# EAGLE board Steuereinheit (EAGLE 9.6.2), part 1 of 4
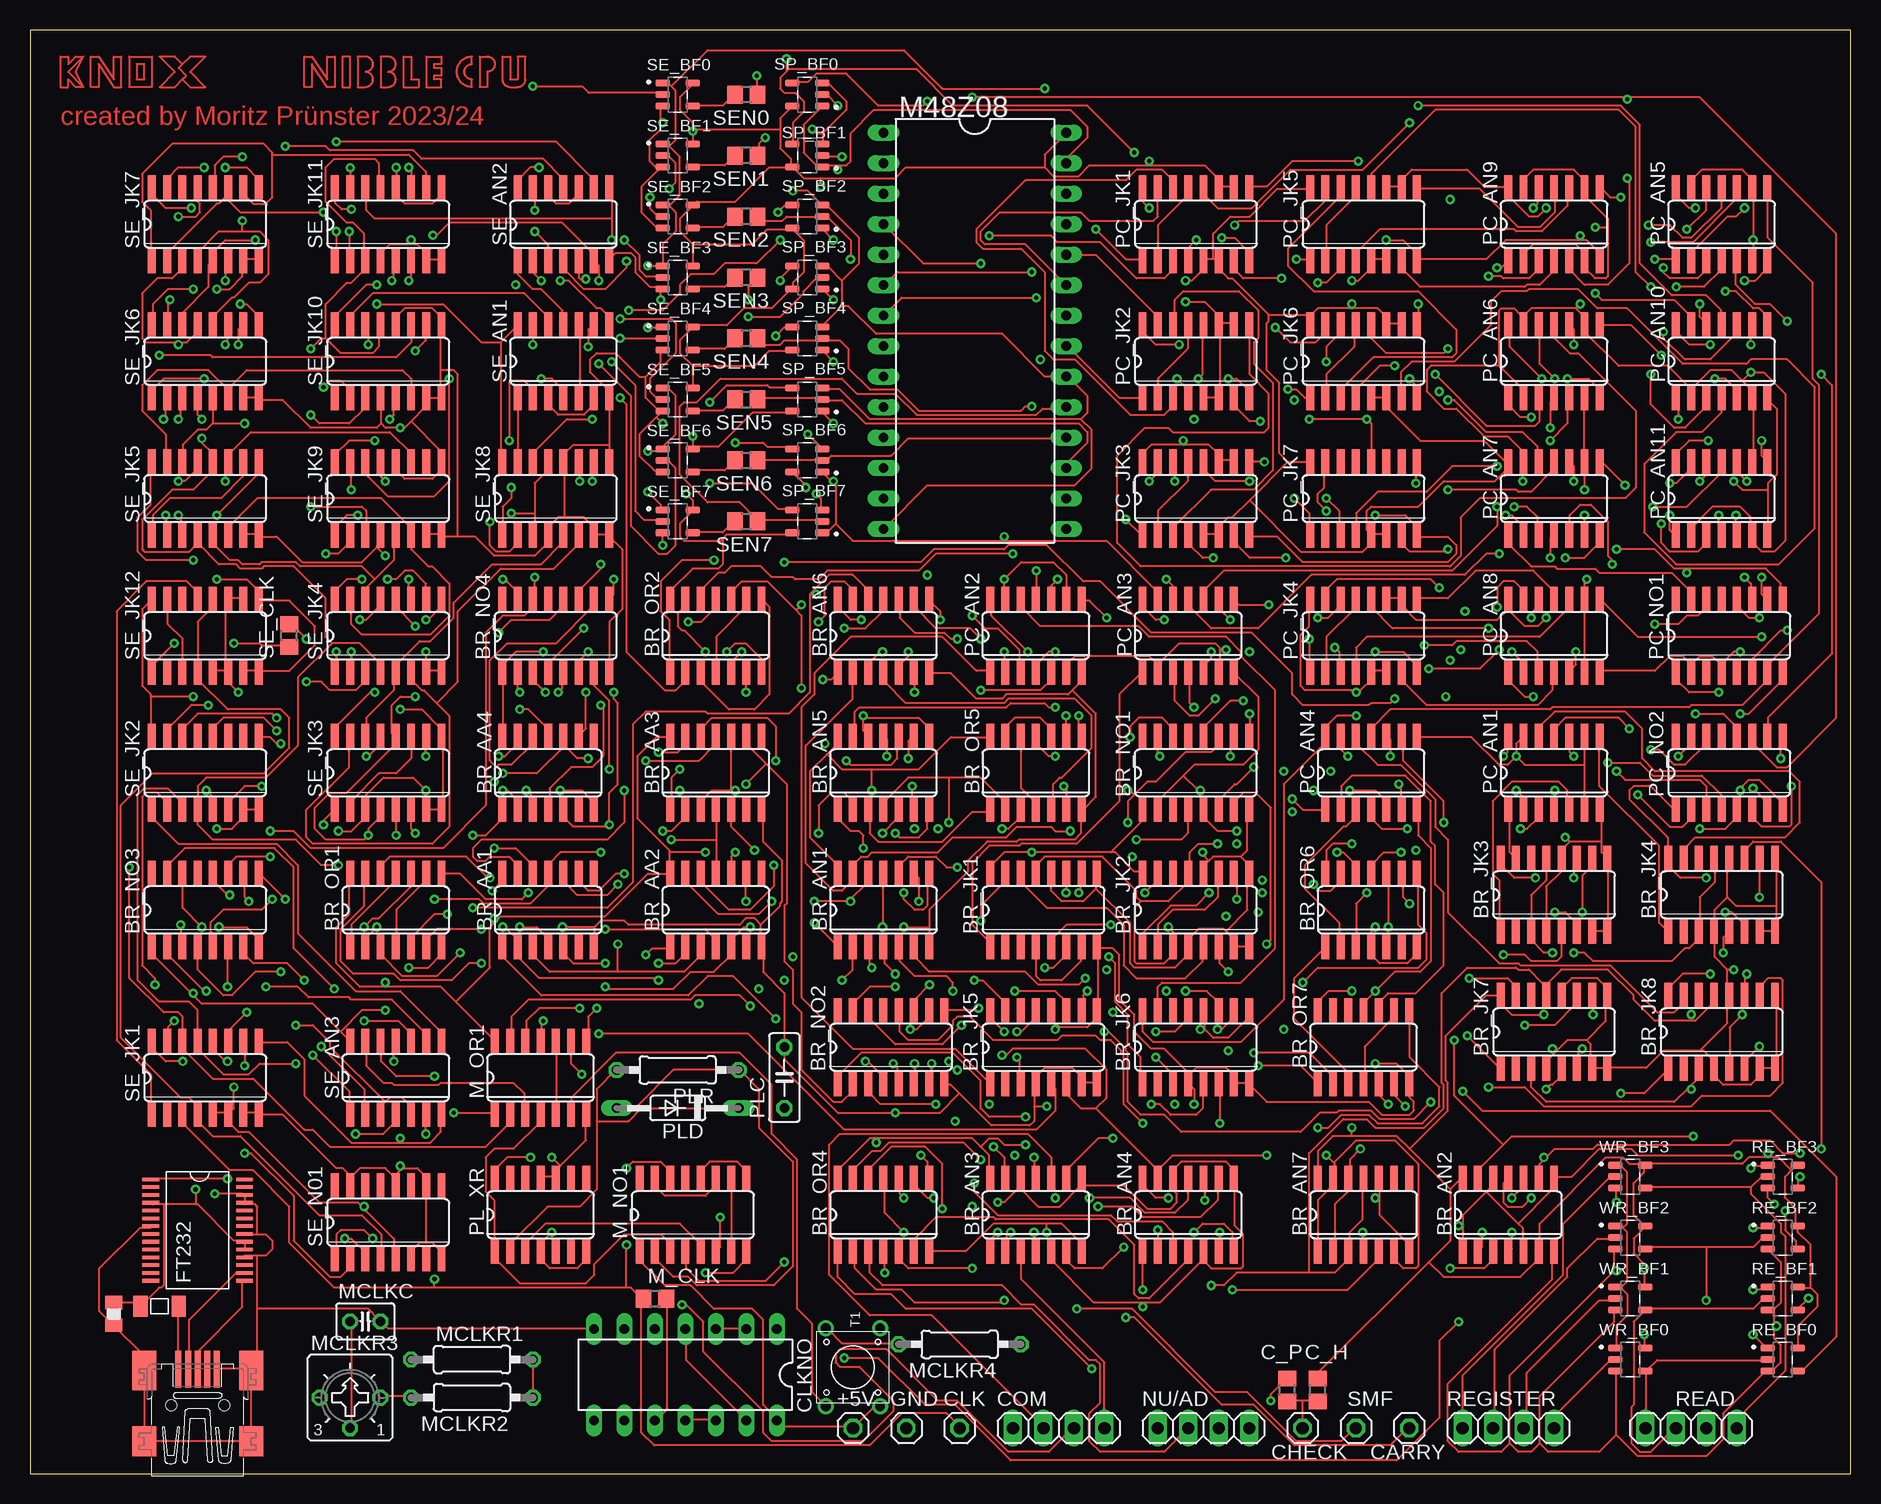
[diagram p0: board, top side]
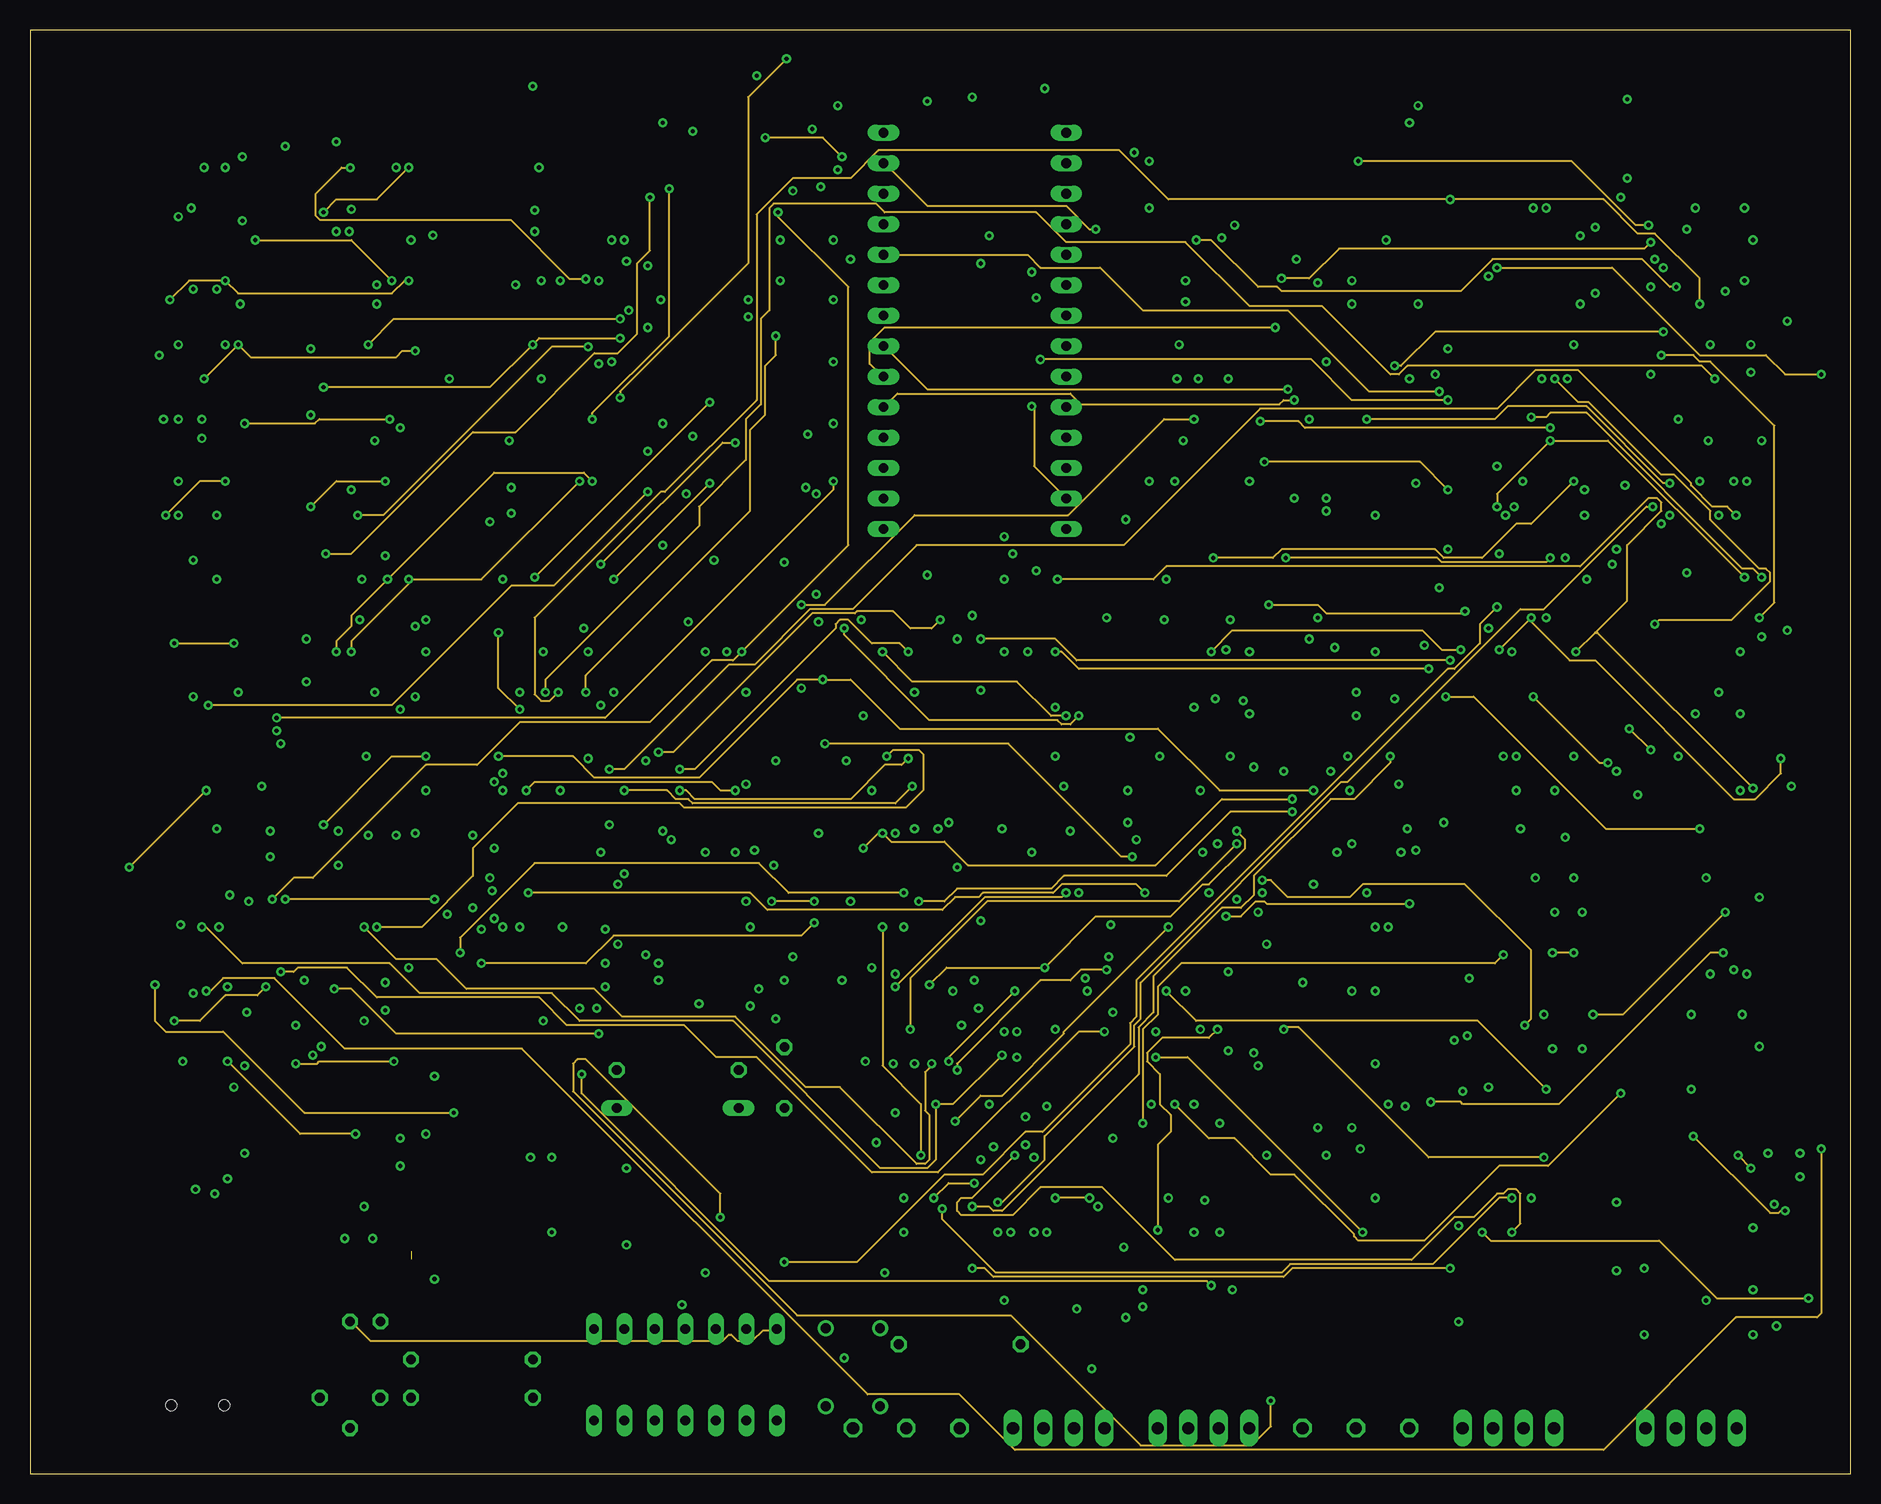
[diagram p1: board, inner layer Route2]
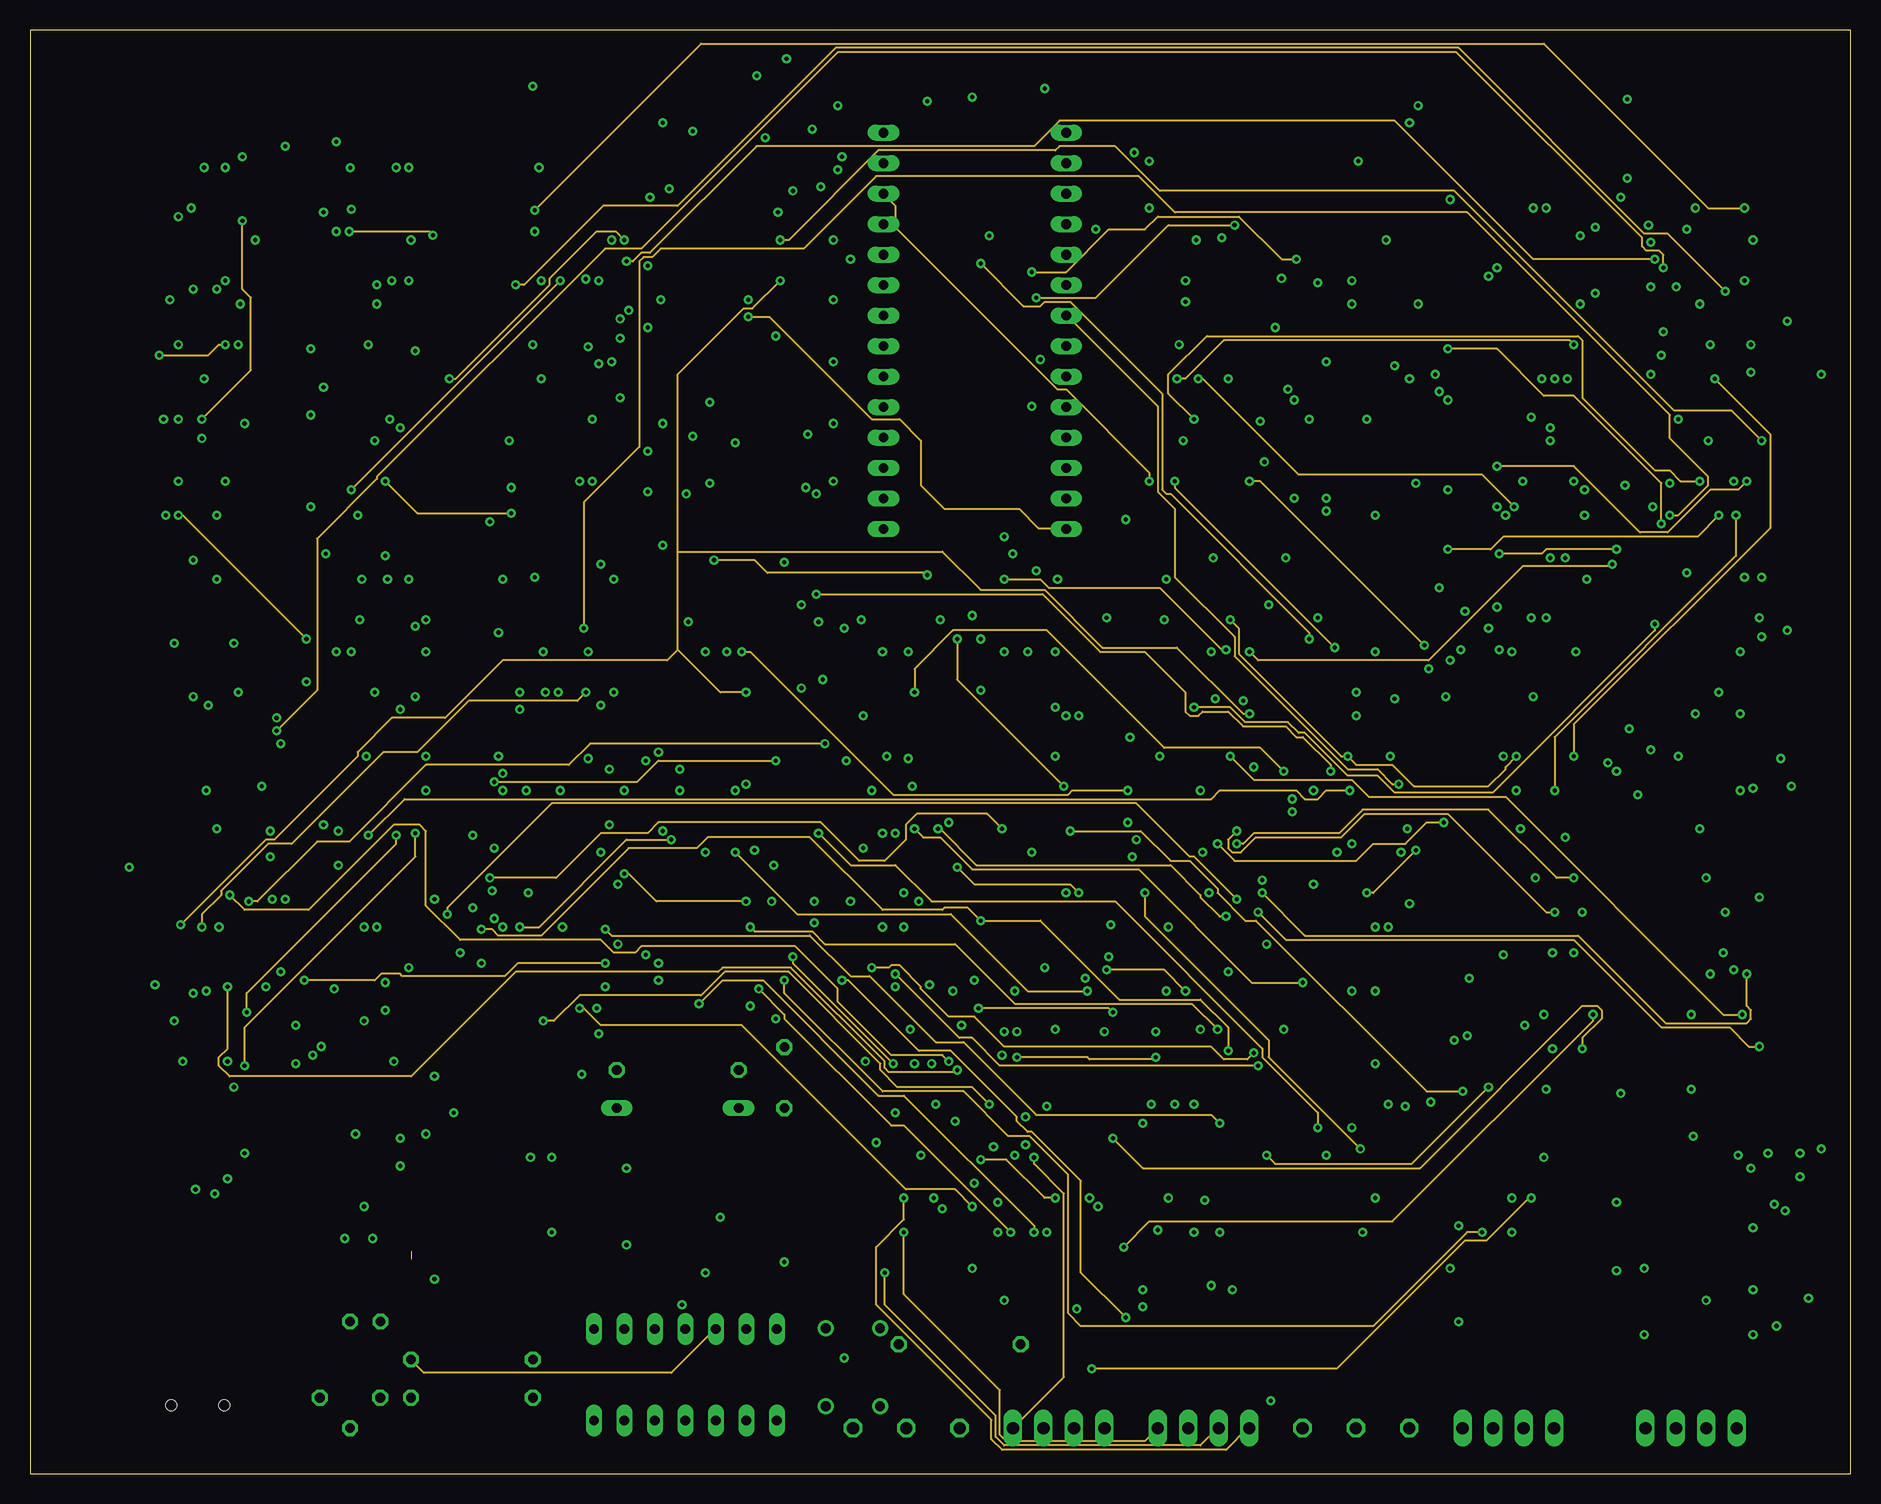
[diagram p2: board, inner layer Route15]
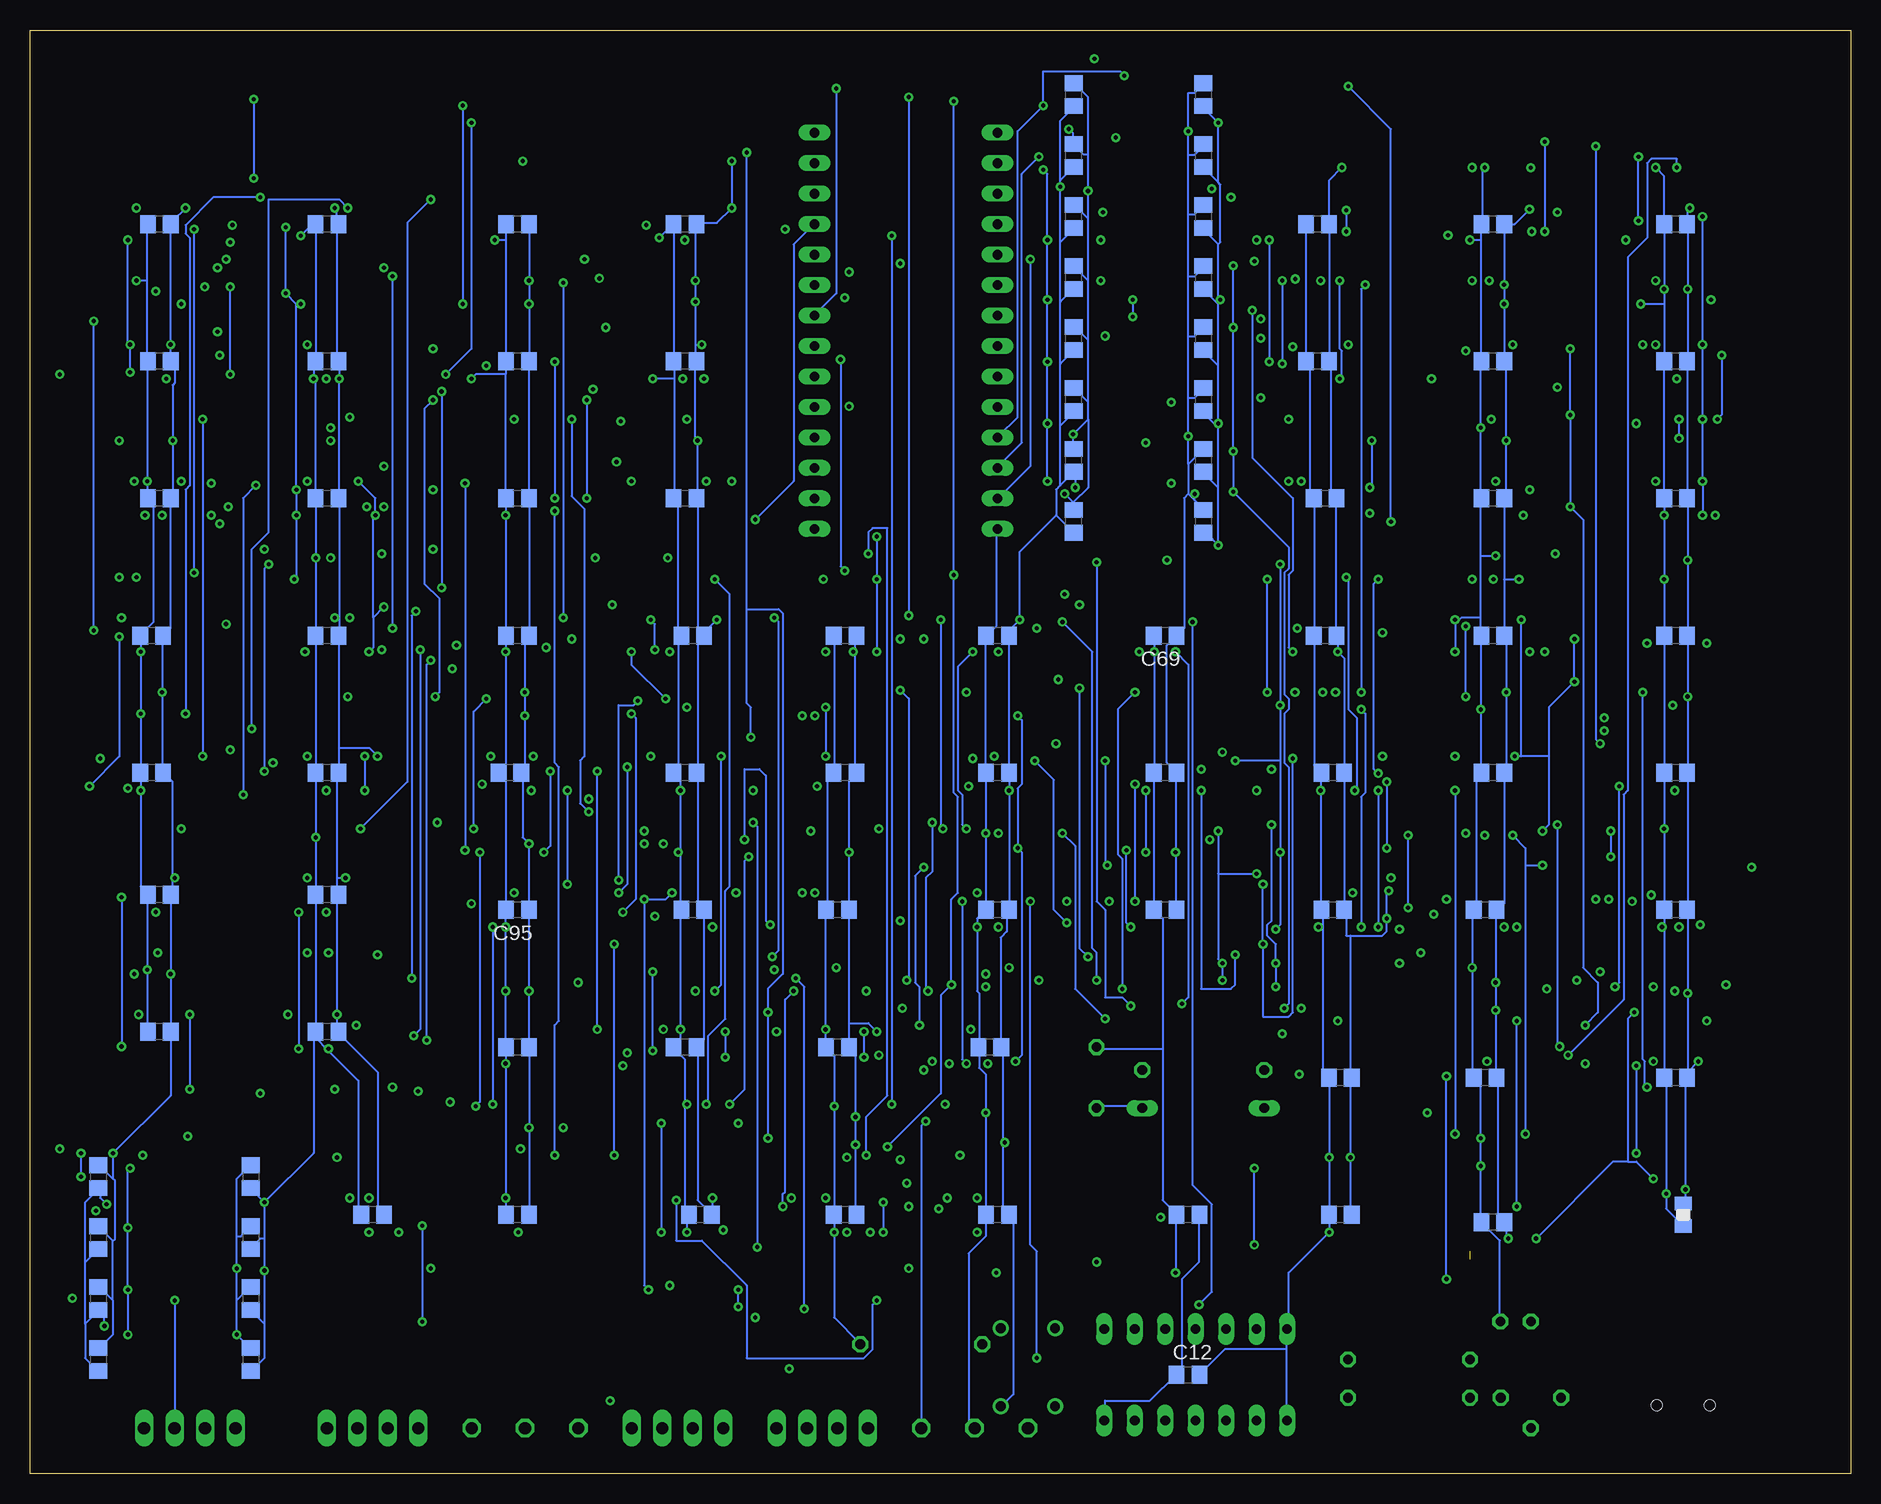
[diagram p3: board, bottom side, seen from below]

Size 151.75 x 120.32 mm. Coordinates in mm from the lower left corner, seen from the top.
Outline: 0,0 151.75,0 151.75,120.32 0,120.32 0,0
Copper layers (1+2*15+16): Top 0.035mm / dielectric 0.2104mm / Route2 0.0175mm / dielectric 1.065mm / Route15 0.0175mm / dielectric 0.2104mm / Bottom 0.035mm
Design rules "default *": minimum track width 6mil, minimum drill 0.35mm, track to track 8mil, track to pad 10mil, pad to pad 8mil, via to via 8mil, smd to smd 6mil, copper to edge 40mil, drill to drill 8mil, minimum pad ring 10mil, minimum via ring 8mil, stop-mask expansion 4mil, vias tented up to drill 0mil, thermal gap 10mil

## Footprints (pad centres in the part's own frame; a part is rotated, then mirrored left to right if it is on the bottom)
1X01 = drill 1.016 octagon: 1 0,0
SO14 = smd 0.66 x 2.032: 1 -3.81,-3.073; 2 -2.54,-3.073; 3 -1.27,-3.073; 4 0,-3.073; 5 1.27,-3.073; 6 2.54,-3.073; 7 3.81,-3.073; 8 3.81,3.073; 9 2.54,3.073; 10 1.27,3.073; 11 0,3.073; 12 -1.27,3.073; 13 -2.54,3.073; 14 -3.81,3.073
SO16 = smd 0.66 x 2.032: 1 -4.445,-3.073; 2 -3.175,-3.073; 3 -1.905,-3.073; 4 -0.635,-3.073; 5 0.635,-3.073; 6 1.905,-3.073; 7 3.175,-3.073; 8 4.445,-3.073; 9 4.445,3.073; 10 3.175,3.073; 11 1.905,3.073; 12 0.635,3.073; 13 -0.635,3.073; 14 -1.905,3.073; 15 -3.175,3.073; 16 -4.445,3.073
C0805 = smd 1.3 x 1.5: 1 -0.95,0; 2 0.95,0
0805F = smd 1.118 x 1.422: 1 -0.953,0; 2 0.953,0
R0805 = smd 1.3 x 1.5: 1 -0.95,0; 2 0.95,0
DIL14 = drill 0.813 long: 1 -7.62,-3.81; 2 -5.08,-3.81; 3 -2.54,-3.81; 4 0,-3.81; 5 2.54,-3.81; 6 5.08,-3.81; 7 7.62,-3.81; 8 7.62,3.81; 9 5.08,3.81; 10 2.54,3.81; 11 0,3.81; 12 -2.54,3.81; 13 -5.08,3.81; 14 -7.62,3.81
1X04 = drill 1.016 long: 1 -3.81,0; 2 -1.27,0; 3 1.27,0; 4 3.81,0
SSOP28 = smd 1.4 x 0.3: 1 -3.9,4.225; 2 -3.9,3.575; 3 -3.9,2.925; 4 -3.9,2.275; 5 -3.9,1.625; 6 -3.9,0.975; 7 -3.9,0.325; 8 -3.9,-0.325; 9 -3.9,-0.975; 10 -3.9,-1.625; 11 -3.9,-2.275; 12 -3.9,-2.925; 13 -3.9,-3.575; 14 -3.9,-4.225; 15 3.9,-4.225; 16 3.9,-3.575; 17 3.9,-2.925; 18 3.9,-2.275; 19 3.9,-1.625; 20 3.9,-0.975; 21 3.9,-0.325; 22 3.9,0.325; 23 3.9,0.975; 24 3.9,1.625; 25 3.9,2.275; 26 3.9,2.925; 27 3.9,3.575; 28 3.9,4.225
DIL28-6 = drill 0.813 long: 1 -16.51,-7.62; 2 -13.97,-7.62; 3 -11.43,-7.62; 4 -8.89,-7.62; 5 -6.35,-7.62; 6 -3.81,-7.62; 7 -1.27,-7.62; 8 1.27,-7.62; 9 3.81,-7.62; 10 6.35,-7.62; 11 8.89,-7.62; 12 11.43,-7.62; 13 13.97,-7.62; 14 16.51,-7.62; 15 16.51,7.62; 16 13.97,7.62; 17 11.43,7.62; 18 8.89,7.62; 19 6.35,7.62; 20 3.81,7.62; 21 1.27,7.62; 22 -1.27,7.62; 23 -3.81,7.62; 24 -6.35,7.62; 25 -8.89,7.62; 26 -11.43,7.62; 27 -13.97,7.62; 28 -16.51,7.62
C025-030X050 = drill 0.813 octagon: 1 -1.27,0; 2 1.27,0
0207/10 = drill 0.813 octagon: 1 -5.08,0; 2 5.08,0
CT6 = drill 0.813 octagon: A 2.515,0; E -2.515,0; S 0,-2.54
C050-025X075 = drill 0.813 octagon: 1 -2.54,0; 2 2.54,0
DO35-10 = drill 0.813 long: A 5.08,0; C -5.08,0
1206 = smd 1.168 x 1.727: 1 -1.587,0; 2 1.587,0
SOT95P280X145-5N = smd 1.21 x 0.59: 1 -1.255,0.95; 2 -1.255,0; 3 -1.255,-0.95; 4 1.255,-0.95; 5 1.255,0.95
TASTE_THT = drill 0.813: A1 -3.251,2.261; A2 3.251,2.261; B1 -3.251,-2.261; B2 3.251,-2.261
32005-201 = smd 3.1 x 0.5: 1 3,1.6; 2 3,0.8; 3 3,0; 4 3,-0.8; 5 3,-1.6 | smd 2.5 x 2: M1 -3,-4.45; M2 -3,4.45 | smd 3.3 x 2: M3 2.9,4.45; M4 2.9,-4.45 | hole 0.9: 0,2.2; 0,-2.2

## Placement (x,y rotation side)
+5V  [1X01]  68.58,3.81 0 top
BR_AA1  4082D  [SO14]  43.18,46.99 0 top
BR_AA2  4082D  [SO14]  57.15,46.99 0 top
BR_AA3  4082D  [SO14]  57.15,58.42 0 top
BR_AA4  4082D  [SO14]  43.18,58.42 0 top
BR_AN1  4081D  [SO14]  71.12,46.99 0 top
BR_AN2  4081D  [SO14]  123.19,21.59 0 top
BR_AN3  4081D  [SO14]  83.82,21.59 0 top
BR_AN4  4081D  [SO14]  96.52,21.59 0 top
BR_AN5  4081D  [SO14]  71.12,58.42 0 top
BR_AN6  4081D  [SO14]  71.12,69.85 0 top
BR_AN7  4081D  [SO14]  111.12,21.59 0 top
BR_JK1  4027D  [SO16]  84.45,46.99 0 top
BR_JK2  4027D  [SO16]  97.16,46.99 0 top
BR_JK3  4027D  [SO16]  127,48.26 0 top
BR_JK4  4027D  [SO16]  140.97,48.26 0 top
BR_JK5  4027D  [SO16]  84.45,35.56 0 top
BR_JK6  4027D  [SO16]  97.16,35.56 0 top
BR_JK7  4027D  [SO16]  127,36.83 0 top
BR_JK8  4027D  [SO16]  140.97,36.83 0 top
BR_NO1  4049D  [SO16]  97.16,58.42 0 top
BR_NO2  4049D  [SO16]  71.75,35.56 0 top
BR_NO3  4049D  [SO16]  14.61,46.99 0 top
BR_NO4  4049D  [SO16]  43.81,69.85 0 top
BR_OR1  4071D  [SO14]  30.48,46.99 0 top
BR_OR2  4071D  [SO14]  57.15,69.85 0 top
BR_OR4  4071D  [SO14]  71.12,21.59 0 top
BR_OR5  4071D  [SO14]  83.82,58.42 0 top
BR_OR6  4071D  [SO14]  111.76,46.99 0 top
BR_OR7  4071D  [SO14]  111.12,35.56 0 top
C1  [C0805]  71.12,46.99 180 bottom
C2  [C0805]  83.82,58.42 180 bottom
C3  [C0805]  42.55,21.59 180 bottom
C4  [C0805]  55.24,21.59 180 bottom
C5  [C0805]  83.82,21.59 180 bottom
C6  [C0805]  95.89,21.59 180 bottom
C7  [C0805]  111.76,58.42 180 bottom
C8  [C0805]  127,48.26 180 bottom
C9  100nF  [0805F]  6.99,13.34 90 top
C10  100nF  [0805F]  13.97,21.59 90 bottom
C11  [C0805]  57.15,58.42 180 bottom
C12  [C0805]  55.24,8.26 0 bottom
C13  [C0805]  29.84,20.96 180 bottom
C14  [C0805]  14.61,33.02 180 bottom
C15  [C0805]  14.61,58.42 180 bottom
C16  [C0805]  30.48,33.02 180 bottom
C17  [C0805]  14.61,104.14 180 bottom
C18  [C0805]  14.61,92.71 180 bottom
C19  [C0805]  97.16,92.71 180 bottom
C20  [C0805]  111.12,92.71 180 bottom
C21  [C0805]  127,69.85 180 bottom
C22  [C0805]  127,81.28 180 bottom
C23  [C0805]  127,92.71 180 bottom
C24  [C0805]  140.97,92.71 180 bottom
C25  [C0805]  140.97,81.28 180 bottom
C26  [C0805]  141.61,69.85 180 bottom
C27  [C0805]  141.61,58.42 180 bottom
C28  [C0805]  140.97,104.14 180 bottom
C29  [C0805]  127,104.14 180 bottom
C30  [C0805]  111.12,104.14 180 bottom
C31  [C0805]  29.84,81.28 180 bottom
C32  [C0805]  14.61,69.85 180 bottom
C33  [C0805]  29.84,69.85 180 bottom
C34  [C0805]  111.12,21.59 180 bottom
C35  [C0805]  14.61,46.99 180 bottom
C36  [C0805]  64.77,79.38 90 bottom
C37  [C0805]  64.77,99.69 90 bottom
C38  [C0805]  64.77,94.62 90 bottom
C39  [C0805]  64.77,89.53 90 bottom
C40  [C0805]  64.77,84.46 90 bottom
C41  [C0805]  133.35,19.68 270 bottom
C42  [C0805]  146.05,24.77 270 bottom
C43  [C0805]  43.81,69.85 180 bottom
C44  [C0805]  71.12,69.85 180 bottom
C45  [C0805]  84.45,46.99 180 bottom
C46  [C0805]  71.75,35.56 180 bottom
C47  [C0805]  84.45,35.56 180 bottom
C48  [C0805]  97.16,58.42 180 bottom
C49  [C0805]  97.16,81.28 180 bottom
C50  [C0805]  96.52,69.85 180 bottom
C51  [C0805]  111.12,81.28 180 bottom
C52  [C0805]  140.97,36.83 180 bottom
C53  [C0805]  140.97,48.26 180 bottom
C54  [C0805]  127,58.42 180 bottom
C55  [C0805]  29.84,104.14 180 bottom
C56  [C0805]  29.84,92.71 180 bottom
C57  [C0805]  43.81,81.28 180 bottom
C58  [C0805]  64.77,104.78 90 bottom
C59  [C0805]  53.98,79.38 270 bottom
C60  [C0805]  53.98,84.46 270 bottom
C61  [C0805]  53.98,89.53 270 bottom
C62  [C0805]  53.98,99.69 270 bottom
C63  [C0805]  53.98,104.78 270 bottom
C64  [C0805]  133.35,9.53 270 bottom
C65  [C0805]  133.35,24.77 270 bottom
C66  [C0805]  146.05,19.68 270 bottom
C67  [C0805]  43.18,46.99 180 bottom
C68  [C0805]  43.18,58.42 180 bottom
C69  [C0805]  57.15,69.85 180 bottom
C70  [C0805]  71.12,58.42 180 bottom
C71  [C0805]  83.82,69.85 180 bottom
C72  [C0805]  42.55,33.02 180 bottom
C73  [C0805]  71.12,21.59 180 bottom
C74  [C0805]  97.16,35.56 180 bottom
C75  [C0805]  96.52,46.99 180 bottom
C76  [C0805]  111.12,69.85 180 bottom
C77  [C0805]  127,36.83 180 bottom
C78  [C0805]  123.19,21.59 180 bottom
C79  [C0805]  97.16,104.14 180 bottom
C80  [C0805]  111.12,35.56 180 bottom
C81  [C0805]  14.61,81.28 180 bottom
C82  [C0805]  44.45,104.14 180 bottom
C83  [C0805]  44.45,92.71 180 bottom
C84  [C0805]  29.84,58.42 180 bottom
C85  [C0805]  64.77,114.94 90 bottom
C86  [C0805]  53.98,114.94 270 bottom
C87  [C0805]  64.77,109.85 90 bottom
C88  [C0805]  53.98,94.62 270 bottom
C89  [C0805]  53.98,109.85 270 bottom
C90  [C0805]  133.35,14.61 270 bottom
C91  [C0805]  146.05,9.53 270 bottom
C92  [C0805]  146.05,14.61 270 bottom
C93  [C0805]  57.15,46.99 180 bottom
C94  [C0805]  30.48,46.99 180 bottom
C95  [C0805]  111.12,46.99 180 bottom
C_H  0  [R0805]  107.31,6.98 90 top
C_P  0  [R0805]  104.77,6.98 90 top
CARRY  [1X01]  114.94,3.81 0 top
CHECK  [1X01]  106.05,3.81 0 top
CLK  [1X01]  77.47,3.81 0 top
CLKNO  40106N  [DIL14]  54.61,8.26 180 top
COM  [1X04]  85.72,3.81 0 top
FT232  [SSOP28]  13.97,20.32 0 top
GND  [1X01]  73.02,3.81 0 top
M48Z08  [DIL28-6]  78.74,95.25 270 top
M_CLK  0  [R0805]  52.07,14.61 0 top
M_NO1  4049D  [SO16]  55.24,21.59 0 top
M_OR1  4071D  [SO14]  42.55,33.02 0 top
MCLKC  [C025-030X050]  27.94,12.7 0 top
MCLKR1  [0207/10]  36.83,9.53 0 top
MCLKR2  [0207/10]  36.83,6.35 180 top
MCLKR3  [CT6]  26.67,6.35 0 top
MCLKR4  [0207/10]  77.47,10.79 180 top
NU/AD  [1X04]  97.79,3.81 0 top
PC_AN1  4081D  [SO14]  127,58.42 0 top
PC_AN2  4081D  [SO14]  83.82,69.85 0 top
PC_AN3  4081D  [SO14]  96.52,69.85 0 top
PC_AN4  4081D  [SO14]  111.76,58.42 0 top
PC_AN5  4081D  [SO14]  140.97,104.14 0 top
PC_AN6  4081D  [SO14]  127,92.71 0 top
PC_AN7  4081D  [SO14]  127,81.28 0 top
PC_AN8  4081D  [SO14]  127,69.85 0 top
PC_AN9  4081D  [SO14]  127,104.14 0 top
PC_AN10  4081D  [SO14]  140.97,92.71 0 top
PC_AN11  4081D  [SO14]  140.97,81.28 0 top
PC_JK1  4027D  [SO16]  97.16,104.14 0 top
PC_JK2  4027D  [SO16]  97.16,92.71 0 top
PC_JK3  4027D  [SO16]  97.16,81.28 0 top
PC_JK4  4027D  [SO16]  111.12,69.85 0 top
PC_JK5  4027D  [SO16]  111.12,104.14 0 top
PC_JK6  4027D  [SO16]  111.12,92.71 0 top
PC_JK7  4027D  [SO16]  111.12,81.28 0 top
PC_NO1  4049D  [SO16]  141.61,69.85 0 top
PC_NO2  4049D  [SO16]  141.61,58.42 0 top
PL_XR  4070D  [SO14]  42.55,21.59 0 top
PLC  [C050-025X075]  62.86,33.02 90 top
PLD  1N4446  [DO35-10]  53.98,30.48 180 top
PLR  [0207/10]  53.98,33.66 180 top
R12  Ferrit  [1206]  10.79,13.97 180 top
RE_BF0  SN74LVC1G126DBVR  [SOT95P280X145-5N]  146.05,9.53 0 top
RE_BF1  SN74LVC1G126DBVR  [SOT95P280X145-5N]  146.05,14.61 0 top
RE_BF2  SN74LVC1G126DBVR  [SOT95P280X145-5N]  146.05,19.68 0 top
RE_BF3  SN74LVC1G126DBVR  [SOT95P280X145-5N]  146.05,24.77 0 top
READ  [1X04]  138.43,3.81 180 top
REGISTER  [1X04]  123.19,3.81 0 top
SE_AN1  4081D  [SO14]  44.45,92.71 0 top
SE_AN2  4081D  [SO14]  44.45,104.14 0 top
SE_AN3  4081D  [SO14]  30.48,33.02 0 top
SE_BF0  SN74LVC1G126DBVR  [SOT95P280X145-5N]  53.98,114.94 0 top
SE_BF1  SN74LVC1G126DBVR  [SOT95P280X145-5N]  53.98,109.85 0 top
SE_BF2  SN74LVC1G126DBVR  [SOT95P280X145-5N]  53.98,104.78 0 top
SE_BF3  SN74LVC1G126DBVR  [SOT95P280X145-5N]  53.98,99.69 0 top
SE_BF4  SN74LVC1G126DBVR  [SOT95P280X145-5N]  53.98,94.62 0 top
SE_BF5  SN74LVC1G126DBVR  [SOT95P280X145-5N]  53.98,89.53 0 top
SE_BF6  SN74LVC1G126DBVR  [SOT95P280X145-5N]  53.98,84.46 0 top
SE_BF7  SN74LVC1G126DBVR  [SOT95P280X145-5N]  53.98,79.38 0 top
SE_CLK  0  [R0805]  21.59,69.85 90 top
SE_JK1  4027D  [SO16]  14.61,33.02 0 top
SE_JK2  4027D  [SO16]  14.61,58.42 0 top
SE_JK3  4027D  [SO16]  29.84,58.42 0 top
SE_JK4  4027D  [SO16]  29.84,69.85 0 top
SE_JK5  4027D  [SO16]  14.61,81.28 0 top
SE_JK6  4027D  [SO16]  14.61,92.71 0 top
SE_JK7  4027D  [SO16]  14.61,104.14 0 top
SE_JK8  4027D  [SO16]  43.81,81.28 0 top
SE_JK9  4027D  [SO16]  29.84,81.28 0 top
SE_JK10  4027D  [SO16]  29.84,92.71 0 top
SE_JK11  4027D  [SO16]  29.84,104.14 0 top
SE_JK12  4027D  [SO16]  14.61,69.85 0 top
SE_N01  4049D  [SO16]  29.84,20.96 0 top
SEN0  0  [R0805]  59.69,114.94 180 top
SEN1  0  [R0805]  59.69,109.85 180 top
SEN2  0  [R0805]  59.69,104.78 180 top
SEN3  0  [R0805]  59.69,99.69 180 top
SEN4  0  [R0805]  59.69,94.62 180 top
SEN5  0  [R0805]  59.69,89.53 0 top
SEN6  0  [R0805]  59.69,84.46 0 top
SEN7  0  [R0805]  59.69,79.38 0 top
SMF  [1X01]  110.49,3.81 0 top
SP_BF0  SN74LVC1G126DBVR  [SOT95P280X145-5N]  64.77,114.94 180 top
SP_BF1  SN74LVC1G126DBVR  [SOT95P280X145-5N]  64.77,109.85 180 top
SP_BF2  SN74LVC1G126DBVR  [SOT95P280X145-5N]  64.77,104.78 180 top
SP_BF3  SN74LVC1G126DBVR  [SOT95P280X145-5N]  64.77,99.69 180 top
SP_BF4  SN74LVC1G126DBVR  [SOT95P280X145-5N]  64.77,94.62 180 top
SP_BF5  SN74LVC1G126DBVR  [SOT95P280X145-5N]  64.77,89.53 180 top
SP_BF6  SN74LVC1G126DBVR  [SOT95P280X145-5N]  64.77,84.46 180 top
SP_BF7  SN74LVC1G126DBVR  [SOT95P280X145-5N]  64.77,79.38 180 top
T1  [TASTE_THT]  68.58,8.89 90 top
WR_BF0  SN74LVC1G126DBVR  [SOT95P280X145-5N]  133.35,9.53 0 top
WR_BF1  SN74LVC1G126DBVR  [SOT95P280X145-5N]  133.35,14.61 0 top
WR_BF2  SN74LVC1G126DBVR  [SOT95P280X145-5N]  133.35,19.68 0 top
WR_BF3  SN74LVC1G126DBVR  [SOT95P280X145-5N]  133.35,24.77 0 top
X2  MINI-USB  [32005-201]  13.97,5.71 90 top

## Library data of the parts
+5V CARRY CHECK CLK COM GND NU/AD READ REGISTER SMF = pinhead
BR_AA1-BR_AA4 BR_AN1-BR_AN7 BR_JK1-BR_JK8 BR_NO1-BR_NO4 BR_OR1 BR_OR2 BR_OR4-BR_OR7 CLKNO M_NO1 M_OR1 PC_AN1-PC_AN11 PC_JK1-PC_JK7 PC_NO1 PC_NO2 PL_XR SE_AN1-SE_AN3 SE_JK1-SE_JK12 SE_N01 = 40xx
C1-C8 C11-C95 MCLKC PLC = rcl; SPICEPREFIX: C
C9 C10 R12 T1 = deto
C_H C_P M_CLK SE_CLK SEN0 SEN1-SEN7 = rcl; SPICEPREFIX: R
FT232 = deto2
M48Z08 = memoryMoritz
MCLKR1 MCLKR2 MCLKR4 PLR = rcl; SPICEPREFIX: L
MCLKR3 = pot
PLD = diode
RE_BF0 RE_BF1-RE_BF3 SE_BF0 SE_BF1-SE_BF7 SP_BF0 SP_BF1-SP_BF7 WR_BF0 WR_BF1-WR_BF3 = SN74LVC1G126DBVR; AVAILABILITY: In Stock; CHECK_PRICES: https://www.snapeda.com/parts/SN74LVC1G126DBVR/Texas+Instruments/view-part/?ref=eda; DESCRIPTION: Single 1.65-V to 5.5-V buffer with 3-state outputs; MF: Texas Instruments; MP: SN74LVC1G126DBVR; PACKAGE: SOT-23-5 Texas Instruments; PRICE: None; PURCHASE-URL: https://www.snapeda.com/api/url_track_click_mouser/?unipart_id=184454&manufacturer=Texas Instruments&part_name=SN74LVC1G126DBVR&search_term=None; SNAPEDA_LINK: https://www.snapeda.com/parts/SN74LVC1G126DBVR/Texas+Instruments/view-part/?ref=snap
X2 = con-cypressindustries; OC_FARNELL: unknown; OC_NEWARK: unknown

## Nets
+5V: +5V.1 BR_AA1.14 BR_AA2.14 BR_AA3.14 BR_AA4.14 BR_AN1.14 BR_AN2.6 BR_AN2.14 BR_AN3.14 BR_AN4.14 BR_AN5.14 BR_AN6.14 BR_AN7.14 BR_JK1.16 BR_JK2.16 BR_JK3.16 BR_JK4.16 BR_JK5.16 BR_JK6.16 BR_JK7.16 BR_JK8.16 BR_NO1.1 BR_NO2.1 BR_NO3.1 BR_NO4.1 BR_OR1.14 BR_OR2.14 BR_OR4.14 BR_OR5.14 BR_OR6.14 BR_OR7.14 C1.1 C2.1 C3.1 C4.1 C5.1 C6.1 C7.1 C8.1 C9.2 C10.2 C11.1 C12.1 C13.1 C14.1 C15.1 C16.1 C17.1 C18.1 C19.1 C20.1 C21.1 C22.1 C23.1 C24.1 C25.1 C26.1 C27.1 C28.1 C29.1 C30.1 C31.1 C32.1 C33.1 C34.1 C35.1 C36.1 C37.1 C38.1 C39.1 C40.1 C41.1 C42.1 C43.1 C44.1 C45.1 C46.1 C47.1 C48.1 C49.1 C50.1 C51.1 C52.1 C53.1 C54.1 C55.1 C56.1 C57.1 C58.1 C59.1 C60.1 C61.1 C62.1 C63.1 C64.1 C65.1 C66.1 C67.1 C68.1 C69.1 C70.1 C71.1 C72.1 C73.1 C74.1 C75.1 C76.1 C77.1 C78.1 C79.1 C80.1 C81.1 C82.1 C83.1 C84.1 C85.1 C86.1 C87.1 C88.1 C89.1 C90.1 C91.1 C92.1 C93.1 C94.1 C95.1 C_H.2 CLKNO.14 FT232.4 FT232.19 FT232.20 M48Z08.28 M_NO1.1 M_OR1.14 PC_AN1.14 PC_AN2.14 PC_AN3.14 PC_AN4.14 PC_AN5.14 PC_AN6.14 PC_AN7.14 PC_AN8.14 PC_AN9.14 PC_AN10.14 PC_AN11.14 PC_JK1.5 PC_JK1.6 PC_JK1.10 PC_JK1.11 PC_JK1.16 PC_JK2.5 PC_JK2.6 PC_JK2.10 PC_JK2.11 PC_JK2.16 PC_JK3.5 PC_JK3.6 PC_JK3.10 PC_JK3.11 PC_JK3.16 PC_JK4.5 PC_JK4.6 PC_JK4.10 PC_JK4.11 PC_JK4.16 PC_JK5.5 PC_JK5.6 PC_JK5.10 PC_JK5.11 PC_JK5.16 PC_JK6.5 PC_JK6.6 PC_JK6.10 PC_JK6.11 PC_JK6.16 PC_JK7.5 PC_JK7.6 PC_JK7.16 PC_NO1.1 PC_NO2.1 PL_XR.14 R12.2 RE_BF0.5 RE_BF1.5 RE_BF2.5 RE_BF3.5 SE_AN1.14 SE_AN2.14 SE_AN3.14 SE_BF0.5 SE_BF1.5 SE_BF2.5 SE_BF3.5 SE_BF4.5 SE_BF5.5 SE_BF6.5 SE_BF7.5 SE_JK1.16 SE_JK2.16 SE_JK3.16 SE_JK4.16 SE_JK5.16 SE_JK6.16 SE_JK7.16 SE_JK8.16 SE_JK9.16 SE_JK10.16 SE_JK11.16 SE_JK12.16 SE_N01.1 SP_BF0.5 SP_BF1.5 SP_BF2.5 SP_BF3.5 SP_BF4.5 SP_BF5.5 SP_BF6.5 SP_BF7.5 T1.B1 WR_BF0.5 WR_BF1.5 WR_BF2.5 WR_BF3.5
BR_CM_N0: BR_AN3.11 COM.1
BR_CM_N1: BR_AN3.10 COM.2
BR_CM_N2: BR_OR2.11 COM.3
BR_CM_N3: BR_AN3.3 COM.4
BR_NR_N0: BR_OR4.11 NU/AD.1
BR_NR_N1: BR_OR4.3 NU/AD.2
BR_NR_N2: BR_OR4.4 NU/AD.3
BR_NR_N3: BR_OR4.10 NU/AD.4
BR_READ: BR_AA2.13 BR_AN1.12 BR_AN2.1 BR_AN2.5 BR_AN2.8 BR_AN2.12 RE_BF0.1 RE_BF1.1 RE_BF2.1 RE_BF3.1
BR_SET: BR_AN7.3 BR_AN7.11 BR_JK7.3 BR_JK7.13 BR_JK8.3 BR_JK8.13 M_OR1.9
BR_SET_N0: BR_JK3.1 PC_AN1.5
BR_SET_N1: BR_JK3.15 PC_AN1.1
BR_SET_N2: BR_JK4.1 PC_AN1.8
BR_SET_N3: BR_JK4.15 PC_AN1.12
BR_SET_N4: BR_JK5.1 PC_AN2.1
BR_SET_N5: BR_JK5.15 PC_AN2.5
BR_SET_N6: BR_JK6.1 PC_AN2.8
BR_SET_N7: BR_JK6.15 PC_AN2.12
BR_SET_N8: BR_JK1.1 PC_AN3.1
BR_SET_N9: BR_JK7.1 PC_AN3.5
BR_SET_N10: BR_JK7.15 PC_AN3.8
BR_SET_N11: BR_JK8.1 PC_AN3.12
BR_SET_N12: BR_JK8.15 PC_AN4.12
GND: BR_AA1.7 BR_AA2.7 BR_AA3.7 BR_AA4.7 BR_AN1.7 BR_AN2.7 BR_AN3.7 BR_AN4.7 BR_AN5.7 BR_AN6.7 BR_AN7.7 BR_AN7.10 BR_JK1.8 BR_JK1.9 BR_JK1.12 BR_JK2.4 BR_JK2.7 BR_JK2.8 BR_JK2.9 BR_JK2.12 BR_JK3.4 BR_JK3.7 BR_JK3.8 BR_JK3.9 BR_JK3.12 BR_JK4.4 BR_JK4.7 BR_JK4.8 BR_JK4.9 BR_JK4.12 BR_JK5.4 BR_JK5.7 BR_JK5.8 BR_JK5.9 BR_JK5.12 BR_JK6.4 BR_JK6.7 BR_JK6.8 BR_JK6.9 BR_JK6.12 BR_JK7.4 BR_JK7.7 BR_JK7.8 BR_JK7.9 BR_JK7.12 BR_JK8.4 BR_JK8.7 BR_JK8.8 BR_JK8.9 BR_JK8.12 BR_NO1.2 BR_NO1.8 BR_NO2.8 BR_NO3.8 BR_NO4.8 BR_OR1.7 BR_OR2.7 BR_OR4.7 BR_OR5.7 BR_OR6.4 BR_OR6.7 BR_OR7.7 BR_OR7.11 C1.2 C2.2 C3.2 C4.2 C5.2 C6.2 C7.2 C8.2 C9.1 C10.1 C11.2 C12.2 C13.2 C14.2 C15.2 C16.2 C17.2 C18.2 C19.2 C20.2 C21.2 C22.2 C23.2 C24.2 C25.2 C26.2 C27.2 C28.2 C29.2 C30.2 C31.2 C32.2 C33.2 C34.2 C35.2 C36.2 C37.2 C38.2 C39.2 C40.2 C41.2 C42.2 C43.2 C44.2 C45.2 C46.2 C47.2 C48.2 C49.2 C50.2 C51.2 C52.2 C53.2 C54.2 C55.2 C56.2 C57.2 C58.2 C59.2 C60.2 C61.2 C62.2 C63.2 C64.2 C65.2 C66.2 C67.2 C68.2 C69.2 C70.2 C71.2 C72.2 C73.2 C74.2 C75.2 C76.2 C77.2 C78.2 C79.2 C80.2 C81.2 C82.2 C83.2 C84.2 C85.2 C86.2 C87.2 C88.2 C89.2 C90.2 C91.2 C92.2 C93.2 C94.2 C95.2 CLKNO.7 CLKNO.8 FT232.7 FT232.18 FT232.21 FT232.25 FT232.26 GND.1 M48Z08.14 M48Z08.20 M_NO1.8 M_OR1.7 MCLKC.2 MCLKR4.1 PC_AN1.7 PC_AN2.7 PC_AN3.7 PC_AN4.7 PC_AN5.7 PC_AN6.7 PC_AN7.7 PC_AN8.7 PC_AN9.7 PC_AN10.7 PC_AN11.7 PC_JK1.8 PC_JK2.8 PC_JK3.8 PC_JK4.8 PC_JK5.8 PC_JK6.8 PC_JK7.8 PC_NO1.2 PC_NO1.4 PC_NO1.8 PC_NO2.8 PL_XR.4 PL_XR.7 PL_XR.10 PL_XR.11 PLC.2 RE_BF0.3 RE_BF1.3 RE_BF2.3 RE_BF3.3 SE_AN1.7 SE_AN2.7 SE_AN3.7 SE_BF0.3 SE_BF1.3 SE_BF2.3 SE_BF3.3 SE_BF4.3 SE_BF5.3 SE_BF6.3 SE_BF7.3 SE_JK1.7 SE_JK1.8 SE_JK1.9 SE_JK2.7 SE_JK2.8 SE_JK3.7 SE_JK3.8 SE_JK3.9 SE_JK4.7 SE_JK4.8 SE_JK4.9 SE_JK5.7 SE_JK5.8 SE_JK5.9 SE_JK6.7 SE_JK6.8 SE_JK6.9 SE_JK7.7 SE_JK7.8 SE_JK7.9 SE_JK8.4 SE_JK8.7 SE_JK8.8 SE_JK8.9 SE_JK8.12 SE_JK9.4 SE_JK9.7 SE_JK9.8 SE_JK9.9 SE_JK9.12 SE_JK10.4 SE_JK10.7 SE_JK10.8 SE_JK10.9 SE_JK10.12 SE_JK11.4 SE_JK11.7 SE_JK11.8 SE_JK11.9 SE_JK11.12 SE_JK12.7 SE_JK12.8 SE_JK12.9 SE_N01.6 SE_N01.8 SE_N01.10 SE_N01.12 SE_N01.15 SP_BF0.3 SP_BF1.3 SP_BF2.3 SP_BF3.3 SP_BF4.3 SP_BF5.3 SP_BF6.3 SP_BF7.3 WR_BF0.3 WR_BF1.3 WR_BF2.3 WR_BF3.3 X2.5 X2.M1 X2.M2 X2.M3 X2.M4
GND2: BR_JK1.4 BR_JK1.7
M_CARRYFLAG: BR_AN1.2 CARRY.1
M_CLK: BR_JK1.13 BR_JK2.3 BR_JK2.13 CLK.1 M_CLK.1 M_NO1.14 PC_AN4.9 SE_AN3.12 SE_JK1.3
M_PC_SET: M_NO1.4 PC_AN5.6 PC_AN5.9 PC_AN5.13 PC_AN6.2 PC_AN6.6 PC_AN6.9 PC_AN6.13 PC_AN7.2 PC_AN7.6 PC_AN7.9 PC_AN7.13 PC_AN8.2 PC_AN8.6 PC_AN8.9 PC_AN8.13 PC_AN9.2 PC_AN9.6 PC_AN9.9 PC_AN9.13 PC_AN10.2 PC_AN10.6 PC_AN10.9 PC_AN10.13 PC_AN11.2 PC_AN11.6 PC_AN11.9
M_RE_N0: BR_AN2.9 BR_AN6.6 RE_BF3.4
M_RE_N1: BR_AN2.13 BR_AN6.9 RE_BF2.4
M_RE_N2: BR_AN2.2 BR_AN6.13 RE_BF1.4
M_RE_N3: BR_AN1.13 BR_AN6.2 RE_BF0.4
M_SAMEFLAG: BR_AN1.6 SMF.1
M_SETPCN0: BR_NO4.7 PC_AN1.4 PC_AN11.5
M_SETPCN1: BR_NO4.5 PC_AN1.3 PC_AN10.12
M_SETPCN2: BR_NO4.3 PC_AN1.10 PC_AN10.5
M_SETPCN3: PC_AN1.11 PC_AN9.12 PC_NO2.14
M_SETPCN4: PC_AN2.3 PC_AN9.5 PC_NO2.11
M_SETPCN5: PC_AN2.4 PC_AN8.12 PC_NO2.9
M_SETPCN6: PC_AN2.10 PC_AN8.5 PC_NO2.7
M_SETPCN7: PC_AN2.11 PC_AN7.12 PC_NO2.5
M_SETPCN8: PC_AN3.3 PC_AN7.5 PC_NO2.3
M_SETPCN9: PC_AN3.4 PC_AN6.12 PC_NO1.14
M_SETPCN10: PC_AN3.10 PC_AN6.5 PC_NO1.11
M_SETPCN11: PC_AN3.11 PC_AN5.12 PC_NO1.9
M_SETPCN12: PC_AN4.11 PC_AN5.8 PC_NO1.7
M_USBDM: FT232.16 X2.2
M_USBDP: FT232.15 X2.3
N$1: SE_AN3.9 SE_JK1.15 SE_JK2.6
N$2: FT232.1 SE_JK1.11 SE_JK3.5 SE_N01.3
N$3: SE_JK1.10 SE_JK3.6 SE_N01.2
N$4: SE_JK1.1 SE_JK12.13
N$5: SE_AN3.2 SE_JK3.1 SE_JK3.10
N$6: SE_JK3.2 SE_JK3.11
N$7: M_OR1.3 SE_AN3.13
N$8: SE_JK4.15 SE_JK5.6 SE_JK9.6
N$9: SE_JK4.14 SE_JK5.5 SE_JK9.5
N$10: SE_JK9.10
N$11: SE_JK5.2 SE_JK5.11 SE_JK9.11
N$12: SE_JK5.1 SE_JK5.10
N$13: SE_JK5.15 SE_JK6.6 SE_JK10.6
N$14: SE_AN1.2 SE_JK8.1
N$15: SE_JK3.15 SE_JK4.6 SE_JK8.6
N$16: SE_JK5.14 SE_JK6.5 SE_JK10.5
N$17: SE_JK6.1 SE_JK6.10 SE_JK10.10
N$18: SE_JK6.14 SE_JK7.5 SE_JK11.5
N$19: SE_JK7.1 SE_JK7.10 SE_JK11.10
N$20: SE_JK6.15 SE_JK7.6 SE_JK11.6
N$21: SE_JK7.2 SE_JK7.11 SE_JK11.11
N$22: SE_AN1.1 SE_JK8.15
N$23: SE_AN1.9 SE_JK9.1
N$24: SE_JK3.14 SE_JK4.5 SE_JK8.5
N$25: SE_JK4.1 SE_JK4.10 SE_JK8.10
N$26: SE_JK4.2 SE_JK4.11 SE_JK8.11
N$27: SE_AN1.8 SE_JK9.15
N$28: SE_AN1.3 SE_AN1.6
N$29: SE_JK6.2 SE_JK6.11 SE_JK10.11
N$30: SE_AN1.5 SE_AN1.10
N$31: SE_AN1.12 SE_JK10.15
N$32: SE_AN3.1 SE_JK7.15
N$33: SE_AN3.3 SE_AN3.5 SE_JK8.3 SE_JK8.13 SE_JK9.3 SE_JK9.13 SE_JK10.3 SE_JK10.13 SE_JK11.3 SE_JK11.13
N$34: SE_AN1.4 SE_AN2.2
N$35: SE_AN1.11 SE_AN2.1
N$36: SE_JK12.3 SE_JK12.15
N$37: SE_JK1.4 SE_JK12.4 SE_JK12.12 SE_N01.4
N$38: M_OR1.2 SE_JK1.14 SE_JK2.5
N$39: SE_AN3.8 SE_JK2.1
N$40: PC_JK1.2 PC_JK1.13
N$41: SE_AN3.11 SE_JK1.13 SE_JK2.3
N$42: M_OR1.1 SE_JK2.2
N$43: SE_AN2.5 SE_JK11.15
N$44: SE_AN2.9 SE_JK11.1
N$45: PC_AN5.2 SE_AN2.3 SE_AN2.13
N$46: SE_AN2.10 SE_AN2.12
N$47: SE_AN2.11 SE_JK2.9
N$48: PC_AN5.1 SE_AN2.4
N$49: PC_AN5.3 SE_JK2.12
N$50: PC_JK1.14 PC_JK2.3
N$51: PC_JK2.2 PC_JK2.13
N$52: PC_JK2.14 PC_JK3.3
N$53: PC_JK3.2 PC_JK3.13
N$54: PC_JK3.14 PC_JK4.3
N$55: PC_JK4.2 PC_JK4.13
N$56: PC_JK4.14 PC_JK5.3
N$57: PC_JK5.2 PC_JK5.13
N$58: PC_JK5.14 PC_JK6.3
N$59: PC_JK6.2 PC_JK6.13
N$60: PC_JK6.14 PC_JK7.3
N$61: BR_NO2.5 BR_OR2.10 PC_AN11.12
N$62: PC_AN5.10 PC_JK1.7
N$63: PC_AN5.4 PC_JK1.4
N$64: PC_AN5.11 PC_JK1.9
N$65: PC_AN6.3 PC_JK1.12
N$66: PC_AN6.4 PC_JK2.7
N$67: PC_AN6.10 PC_JK2.4
N$68: PC_AN6.11 PC_JK2.9
N$69: PC_AN7.3 PC_JK2.12
N$70: PC_AN7.4 PC_JK3.7
N$71: PC_AN7.10 PC_JK3.4
N$72: PC_AN7.11 PC_JK3.9
N$73: PC_AN8.3 PC_JK3.12
N$74: PC_AN8.4 PC_JK4.7
N$75: PC_AN8.10 PC_JK4.4
N$76: PC_AN8.11 PC_JK4.9
N$77: PC_AN9.3 PC_JK4.12
N$78: PC_AN9.4 PC_JK5.7
N$79: PC_AN9.10 PC_JK5.4
N$80: PC_AN9.11 PC_JK5.9
N$81: PC_AN10.3 PC_JK5.12
N$82: PC_AN10.4 PC_JK6.7
N$83: PC_AN10.10 PC_JK6.4
N$84: PC_AN10.11 PC_JK6.9
N$85: PC_AN11.3 PC_JK6.12
N$86: PC_AN11.4 PC_JK7.7
N$87: PC_AN11.10 PC_JK7.4
N$88: PC_AN5.5 PC_NO1.6
N$89: BR_AN1.10 BR_JK1.10 BR_NO2.14
N$90: BR_OR2.4 BR_OR2.9
N$91: PC_AN6.1 PC_NO1.10
N$92: BR_OR2.3 BR_OR2.8
N$93: PC_AN6.8 PC_NO1.12
N$94: BR_AN1.8 BR_OR1.3
N$95: PC_AN7.1 PC_NO1.15
N$96: BR_AN3.4 BR_OR2.13
N$97: PC_AN7.8 PC_NO2.2
N$98: BR_JK1.11 BR_NO2.15
N$99: PC_AN8.1 PC_NO2.4
N$100: BR_AN3.1 BR_AN3.5 BR_AN3.8 BR_AN3.12 BR_AN4.1 BR_AN4.5 BR_AN4.8 BR_AN4.12 PC_AN11.11
N$101: PC_AN8.8 PC_NO2.6
N$102: BR_AN4.11 BR_OR4.13
N$103: PC_AN9.1 PC_NO2.10
N$104: BR_AN4.10 BR_OR4.2
N$105: PC_AN9.8 PC_NO2.12
N$106: BR_AN4.4 BR_OR4.6
N$107: PC_AN10.1 PC_NO2.15
N$108: BR_AN4.3 BR_OR4.9
N$109: BR_NO4.2 PC_AN10.8
N$110: BR_JK6.11 BR_NO3.6
N$111: BR_NO4.4 PC_AN11.1
N$112: BR_OR1.4 BR_OR1.9
N$113: BR_NO4.6 PC_AN11.8
N$114: BR_AN2.4 BR_OR2.12
N$115: BR_JK3.3 BR_JK3.13 BR_JK4.3 BR_JK4.13
N$116: BR_AN2.10 BR_OR4.12
N$117: BR_AN2.11 BR_OR4.1
N$118: BR_AN2.3 BR_OR4.5
N$119: BR_AN1.11 BR_OR4.8
N$120: BR_AA1.12 BR_AA2.12 BR_AA3.12 BR_AA4.12 BR_NO4.10
N$121: BR_AA1.4 BR_AA2.11 BR_AA3.4 BR_AA4.11 BR_NO4.12
N$122: BR_AA1.3 BR_AA1.10 BR_AA2.3 BR_AA4.10 BR_NO4.15
N$123: BR_AA1.2 BR_AA1.9 BR_AA2.2 BR_AA2.9 BR_AA3.2 BR_AA3.9 BR_AA4.2 BR_NO2.2
N$124: BR_JK6.5 BR_NO3.10
N$125: BR_AA1.1 BR_AN5.2 BR_OR7.8
N$126: BR_AA1.13 BR_AN5.6
N$127: BR_AN5.1 BR_AN5.5 BR_AN5.8 BR_AN5.12 BR_NO2.4 PC_AN4.1
N$128: BR_AN1.5 BR_AN5.4 BR_OR5.2
N$129: BR_AN5.3 BR_OR5.1
N$130: BR_AN1.3 BR_OR7.2
N$131: BR_AA2.1 BR_AN5.9
N$132: BR_AN1.1 BR_AN5.10 BR_OR1.13
N$133: BR_AN1.4 BR_OR7.1
N$134: BR_OR1.12 BR_OR5.3
N$135: BR_AA3.1 BR_AN6.5 BR_OR6.8
N$136: BR_AA3.13 BR_AN6.8 BR_OR6.9
N$137: BR_AA4.1 BR_AN6.12 BR_OR6.12
N$138: BR_AA4.13 BR_AN6.1 BR_OR6.13
N$139: BR_AN6.4 BR_OR5.5
N$140: BR_AN6.10 BR_OR5.6
N$141: BR_OR5.4 BR_OR5.12
N$142: BR_OR5.10 BR_OR5.13
N$143: BR_AN6.11 BR_OR5.8
N$144: BR_AN6.3 BR_OR5.9
N$145: BR_AN5.13 BR_OR5.11
N$146: BR_AN5.11 BR_OR1.2
N$147: BR_OR1.1 BR_OR1.11
N$148: BR_JK1.14 BR_JK2.5
N$149: BR_JK5.11 BR_NO3.12
N$150: BR_AN7.4 BR_JK5.3 BR_JK5.13 BR_JK6.3 BR_JK6.13
N$151: BR_JK2.2 BR_JK2.11
N$152: BR_JK5.5 BR_NO3.15
N$153: BR_OR6.3 PC_JK7.9
N$154: BR_AN1.9 BR_NO2.6 PC_AN11.13 PC_JK7.12
N$155: BR_NO2.7 BR_OR1.10
N$156: BR_JK8.11 BR_NO1.6
N$157: BR_JK8.5 BR_NO1.10
N$158: BR_JK7.11 BR_NO1.12
N$159: BR_JK1.15 BR_JK2.6 BR_OR1.6
N$160: BR_JK4.11 BR_NO3.2
N$161: BR_JK4.5 BR_NO3.4
N$162: BR_JK3.11 BR_NO2.10
N$163: BR_JK3.5 BR_NO2.12
N$164: BR_JK7.5 BR_NO1.15
N$165: BR_JK1.3
N$166: BR_JK1.5 BR_NO1.4
N$167: BR_OR6.10 BR_OR7.5
N$168: CLKNO.10 M_CLK.2
N$169: SE_BF7.4 SEN7.1
N$170: SE_BF6.4 SEN6.1
N$171: SE_BF5.4 SEN5.1
N$172: SE_BF4.4 SEN4.2
N$173: SE_BF3.4 SEN3.2
N$174: SE_BF2.4 SEN2.2
N$175: SE_BF1.4 SEN1.2
N$176: SE_BF0.4 SEN0.2
N$177: CLKNO.11 CLKNO.12
N$178: SE_CLK.1 SE_JK12.1
N$179: C_P.2 M_NO1.6
N$180: CLKNO.4 CLKNO.13
N$181: C_H.1 C_P.1 CHECK.1
N$182: MCLKR2.2 MCLKR3.A
N$183: M_NO1.2 PLD.A PLR.1
N$184: PL_XR.2 PLC.1 PLD.C PLR.2
N$185: M_OR1.13 PC_AN4.4
N$186: RE_BF0.2 READ.4 WR_BF0.4
N$187: M_NO1.5 PL_XR.3
N$188: RE_BF1.2 READ.3 WR_BF1.4
N$189: M_OR1.11 PC_JK1.3
N$190: RE_BF2.2 READ.2 WR_BF2.4
N$191: M_OR1.12 PC_AN4.10
N$192: RE_BF3.2 READ.1 WR_BF3.4
N$193: REGISTER.4 WR_BF0.2
N$194: REGISTER.3 WR_BF1.2
N$195: REGISTER.2 WR_BF2.2
N$196: REGISTER.1 WR_BF3.2
N$197: WR_BF0.1 WR_BF1.1 WR_BF2.1 WR_BF3.1
N$198: M_OR1.6 T1.A1
N$199: CLKNO.1 MCLKC.1 MCLKR3.S
N$200: SE_AN2.8 SE_BF7.2 SE_JK11.14
N$201: SE_AN2.6 SE_BF6.2 SE_JK11.2
N$202: SE_BF5.2 SE_JK10.14
N$203: SE_AN1.13 SE_BF4.2 SE_JK10.2
N$204: SE_BF3.2 SE_JK9.14
N$205: SE_BF0.2 SE_JK8.2
N$206: SE_BF1.2 SE_JK8.14
N$207: SE_BF2.2 SE_JK9.2
N$208: M_NO1.11 M_NO1.15
N$209: M_NO1.9 M_NO1.12
N$210: M_NO1.7 M_NO1.10
N$211: CLKNO.2 CLKNO.3 MCLKR1.1
N$212: MCLKR1.2 MCLKR2.1
N$213: BR_OR6.11 BR_OR7.6
N$214: MCLKR4.2 T1.A2
N$215: BR_OR7.4 BR_OR7.9
N$216: BR_OR7.10 PC_AN4.2
N$217: BR_OR6.1 BR_OR7.3
N$218: BR_AN7.5 BR_JK2.1 BR_JK2.10 BR_OR1.5
N$219: BR_AN7.2 BR_AN7.12 BR_JK2.15 BR_OR1.8
N$220: M_OR1.5 M_OR1.10
N$221: BR_OR6.2 PC_AN4.3
N$222: BR_AN7.1 BR_AN7.6 BR_AN7.13 PC_JK7.15
N$223: M_NO1.3 M_OR1.4 PL_XR.1
PC_N0: M48Z08.10 PC_JK7.1
PC_N1: M48Z08.9 PC_JK6.15
PC_N2: M48Z08.8 PC_JK6.1
PC_N3: M48Z08.7 PC_JK5.15
PC_N4: M48Z08.6 PC_JK5.1
PC_N5: M48Z08.5 PC_JK4.15
PC_N6: M48Z08.4 PC_JK4.1
PC_N7: M48Z08.3 PC_JK3.15
PC_N8: M48Z08.25 PC_JK3.1
PC_N9: M48Z08.24 PC_JK2.15
PC_N10: M48Z08.21 PC_JK2.1
PC_N11: M48Z08.23 PC_JK1.15
PC_N12: M48Z08.2 PC_JK1.1
SE_CLK: SE_AN3.6 SE_CLK.2 SE_JK3.3 SE_JK3.13 SE_JK4.3 SE_JK4.13 SE_JK5.3 SE_JK5.13 SE_JK6.3 SE_JK6.13 SE_JK7.3 SE_JK7.13
SE_ENCLK: SE_AN3.10 SE_JK1.5 SE_JK1.6 SE_JK12.5 SE_JK12.6 SE_JK12.10 SE_JK12.11 SE_N01.5
SE_N0: M48Z08.11 SEN0.1 SP_BF0.2
SE_N1: M48Z08.12 SEN1.1 SP_BF1.2
SE_N2: M48Z08.13 SEN2.1 SP_BF2.2
SE_N3: M48Z08.15 SEN3.1 SP_BF3.2
SE_N4: M48Z08.16 SEN4.1 SP_BF4.2
SE_N5: M48Z08.17 SEN5.2 SP_BF5.2
SE_N6: M48Z08.18 SEN6.2 SP_BF6.2
SE_N7: M48Z08.19 SEN7.2 SP_BF7.2
SE_NEWNUMBER: PC_AN4.5 SE_AN3.4 SE_JK1.12 SE_JK2.4 SE_JK3.4 SE_JK3.12 SE_JK4.4 SE_JK4.12 SE_JK5.4 SE_JK5.12 SE_JK6.4 SE_JK6.12 SE_JK7.4 SE_JK7.12
SE_WRITE_N: M48Z08.27 PC_AN1.2 PC_AN1.6 PC_AN1.9 PC_AN1.13 PC_AN2.2 PC_AN2.6 PC_AN2.9 PC_AN2.13 PC_AN3.2 PC_AN3.6 PC_AN3.9 PC_AN3.13 PC_AN4.8 PC_AN4.13 SE_JK2.14 SP_BF0.1 SP_BF1.1 SP_BF2.1 SP_BF3.1 SP_BF4.1 SP_BF5.1 SP_BF6.1 SP_BF7.1
SE_WRITE_P: M48Z08.22 M_OR1.8 PC_AN4.6 SE_BF0.1 SE_BF1.1 SE_BF2.1 SE_BF3.1 SE_BF4.1 SE_BF5.1 SE_BF6.1 SE_BF7.1 SE_JK2.15
SP_N0: BR_AN3.13 BR_JK1.6 BR_JK3.6 BR_NO1.5 BR_NO2.11 BR_OR2.1 SP_BF0.4
SP_N1: BR_AN3.9 BR_JK3.10 BR_JK7.6 BR_NO1.14 BR_NO2.9 BR_OR2.2 SP_BF1.4
SP_N2: BR_AN3.6 BR_JK4.6 BR_JK7.10 BR_NO1.11 BR_NO3.5 BR_OR2.5 SP_BF2.4
SP_N3: BR_AN3.2 BR_JK4.10 BR_JK8.6 BR_NO1.9 BR_NO3.3 BR_OR2.6 SP_BF3.4
SP_N4: BR_AA4.9 BR_AN4.13 BR_JK5.6 BR_JK8.10 BR_NO1.7 BR_NO2.3 BR_NO3.14 SP_BF4.4
SP_N5: BR_AA2.10 BR_AA3.3 BR_AA3.10 BR_AA4.3 BR_AN4.9 BR_JK5.10 BR_NO3.11 BR_NO4.14 SP_BF5.4
SP_N6: BR_AA1.11 BR_AA2.4 BR_AA3.11 BR_AA4.4 BR_AN4.6 BR_JK6.6 BR_NO3.9 BR_NO4.11 SP_BF6.4
SP_N7: BR_AA1.5 BR_AA2.5 BR_AA3.5 BR_AA4.5 BR_AN4.2 BR_JK6.10 BR_NO3.7 BR_NO4.9 SP_BF7.4
USB_4: R12.1 X2.1

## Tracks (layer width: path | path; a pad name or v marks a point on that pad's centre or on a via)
+5V  (via drill 0.35)
  Top 0.152: PC_JK2.5 97.89,89.66 98.96,89.66 PC_JK2.6 99.14,89.66 99.14,95.71 PC_JK2.11 | PC_JK2.11 99.14,95.88 100.2,95.88 PC_JK2.10 | v95.76,94.11 93.8,94.11 92.73,95.17 92.73,95.71 PC_JK2.16 | v93.27,105.49 92.73,106.02 92.73,107.09 PC_JK1.16 | v96.29,97.66 97.89,97.66 98.96,96.6 98.96,95.88 PC_JK2.11 | v94.87,22.99 93.8,22.99 92.73,24.05 92.73,24.59 BR_AN4.14 | 96.11,85.75 98.25,85.75 98.96,85.04 98.96,84.51 PC_JK3.11 99.14,84.51 100.2,84.51 PC_JK3.10 | 96.11,85.75 93.45,85.75 92.73,85.04 92.73,84.51 PC_JK3.16 | v94.51,71.17 93.8,71.17 92.73,72.24 92.73,72.77 PC_AN3.14 | v96.11,86.11 96.11,85.75 | 106.78,96.6 106.78,95.88 PC_JK6.16 106.78,96.6 | 106.78,96.6 107.31,97.13 110.16,97.13 | 110.16,97.13 112.29,97.13 113,96.42 113,95.88 PC_JK6.11 113.18,95.88 114.25,95.88 PC_JK6.10 | 98.6,101.22 98.96,101.22 PC_JK1.6 99.14,101.04 99.14,100.33 99.85,99.62 100.2,99.62 103.23,96.6 | 98.6,101.22 97.89,101.22 PC_JK1.5 97.71,101.04 97.71,100.33 96.83,99.44 v96.29,99.44 | 98.6,101.22 98.6,103.35 100.02,104.78 101.62,104.78 103.94,107.09 106.6,107.09 PC_JK5.16 | 103.23,96.6 106.78,96.6 | PC_JK6.5 111.76,89.66 113,89.66 PC_JK6.6 113.18,89.48 113.18,88.77 115.85,86.11 121.18,86.11 122.78,84.51 123.14,84.51 PC_AN7.14 123.14,84.33 123.14,83.8 122.07,82.73 117.8,82.73 115.67,80.59 111.76,80.59 111.4,80.24 111.4,78.64 111.76,78.28 | 111.76,78.28 113,78.28 PC_JK7.6 | PC_JK3.5 97.89,78.28 98.96,78.28 PC_JK3.6 99.14,78.28 99.14,78.99 99.85,79.7 100.2,79.7 101.62,81.13 | 104.83,84.33 106.6,84.33 PC_JK7.16 | 101.62,81.13 104.83,84.33 | 101.62,81.13 105.89,76.86 111.05,76.86 111.76,77.57 PC_JK7.5 111.76,78.28
  Top 0.152: 103.23,96.6 103.23,96.06 103.05,95.88 103.05,91.97 104.11,90.91 104.11,85.04 104.83,84.33 | BR_JK6.16 92.73,38.63 92.73,36.86 93.62,35.97 100.91,35.97 104.47,39.52 104.47,57.48 107.85,60.86 107.85,61.39 PC_AN4.14 108.03,61.57 108.03,62.28 108.91,63.17 v110.52,63.17 | BR_OR7.14 107.31,39.34 108.2,40.23 v110.16,40.23 | v110.16,52.5 108.56,52.5 108.03,51.97 108.03,50.19 BR_OR6.14 | PC_JK5.6 113,101.22 111.76,101.22 PC_JK5.5 111.76,100.51 110.69,99.44 v110.16,99.44 | PC_JK4.6 113,66.9 111.76,66.9 PC_JK4.5 111.76,66.19 110.87,65.3 110.52,65.3 | 110.52,65.3 106.25,65.3 105.89,65.66 105.89,69.93 106.6,70.64 106.6,72.77 PC_JK4.16 | v110.52,65.13 110.52,65.3 | v110.16,97.49 110.16,97.13 | PC_JK5.11 113.18,107.26 114.25,107.26 PC_JK5.10 114.43,107.26 114.43,107.97 115.14,108.69 119.76,108.69 121.18,107.26 123.14,107.26 PC_AN9.14 123.32,107.09 123.32,106.38 124.92,104.78 125.63,104.78 v126.34,105.49 | v125.98,91.26 123.32,93.93 123.32,95.71 PC_AN6.14 | PC_JK4.11 113.18,72.95 114.25,72.95 PC_JK4.10 114.43,72.77 114.43,72.24 115.49,71.17 122.25,71.17 123.14,72.06 | 123.14,72.06 123.14,72.77 PC_AN8.14 123.14,72.06 | v125.45,49.66 123.67,49.66 122.61,50.72 122.61,51.26 BR_JK3.16 | v122.78,59.79 123.14,60.15 123.14,61.39 PC_AN1.14 | 123.14,72.06 124.56,70.64 125.63,70.64 v126.34,71.35 | v134.52,11.61 134.52,10.54 WR_BF0.5 | WR_BF1.5 134.52,15.7 v134.52,17.12 134.52,17.48 133.63,18.36 133.63,19.61 134.52,20.5 WR_BF2.5 134.52,20.68 133.63,21.57 133.63,24.23 134.52,25.12 134.52,25.65 WR_BF3.5 | 148.39,15.52 148.92,14.99 148.92,13.92 147.32,12.32 147.32,10.54 RE_BF0.5
  Top 0.152: 148.39,15.52 147.32,15.52 RE_BF1.5 | 148.39,15.52 148.39,19.07 147.32,20.14 147.32,20.5 RE_BF2.5 147.14,20.68 147.14,22.1 146.25,22.99 146.25,24.77 146.79,25.3 | 146.79,25.3 147.14,25.65 RE_BF3.5 | 144.83,26.37 145.72,26.37 146.79,25.3 | 144.83,26.37 143.23,26.37 142.7,25.83 134.7,25.83 WR_BF3.5 | 144.83,26.37 v144.83,26.72 | C_H.2 107.31,8.41 116.56,17.65 | 116.56,17.65 118.34,19.43 118.34,23.7 | 118.34,23.7 119.23,24.59 BR_AN2.14 | BR_AN7.14 107.31,26.9 108.56,28.14 110.16,28.14 | 110.16,28.14 113.89,28.14 114.96,27.08 | 118.34,23.7 114.96,27.08 | 114.96,27.08 118.16,30.28 118.16,32.59 117.98,32.77 117.98,36.5 121.36,39.88 122.43,39.88 BR_JK7.16 122.61,39.88 122.61,39.17 123.5,38.28 v126.16,38.28 | 116.56,17.65 117.8,16.41 124.21,16.41 125.63,17.83 125.63,18.36 BR_AN2.6 125.81,18.54 125.81,20.85 131.32,26.37 132.74,26.37 133.27,25.83 134.52,25.83 WR_BF3.5 | v139.85,86.11 138.25,86.11 137.19,85.04 137.19,84.51 PC_AN11.14 | v140.03,94.11 138.25,94.11 137.19,95.17 137.19,95.71 PC_AN10.14 | v138.79,105.49 138.25,105.49 137.19,106.55 137.19,107.09 PC_AN5.14 | v140.74,65.13 138.25,65.13 137.19,66.19 137.19,66.73 PC_NO1.1 | PC_NO2.1 137.01,55.35 135.05,57.3 133.63,57.3 133.27,56.95 133.27,56.24 136.47,53.04 136.47,51.44 BR_JK4.16 136.65,51.26 136.65,50.55 137.54,49.66 v139.68,49.66 | v140.03,41.66 137.72,41.66 136.65,40.59 136.65,40.06 BR_JK8.16 | 110.16,28.14 v110.16,28.85 | 13.44,40.06 14.33,39.17 23.57,39.17 25.88,36.86 | 13.44,40.06 10.24,43.26 10.24,43.79 BR_NO3.1 | 25.88,36.86 26.59,36.14 SE_AN3.14 | C9.2 7.04,14.28 8.99,14.28 9.17,14.1 R12.2 9.35,14.1 10.77,15.52 10.95,15.52 11.12,15.7 11.12,22.45
  Top 0.152: FT232.19 17.88,18.72 17.88,19.25 FT232.20 17.7,19.43 16.99,19.43 13.97,22.45 13.79,22.45 | 13.79,22.45 11.12,22.45 | 11.12,22.45 10.24,22.45 FT232.4 | v13.61,98.73 11.48,98.73 10.24,97.49 10.24,95.88 SE_JK6.16 | v13.44,105.49 11.3,105.49 10.24,106.55 10.24,107.09 SE_JK7.16 | v12.72,34.37 11.3,34.37 10.24,35.43 10.24,35.97 SE_JK1.16 | 10.06,64.77 10.06,64.95 9.35,65.66 9.35,72.06 10.06,72.77 SE_JK12.16 | 10.06,64.77 10.06,61.57 SE_JK2.16 | v13.61,76.15 9.7,76.15 8.99,76.86 8.99,79.7 10.06,80.77 10.06,84.33 SE_JK5.16 | v13.61,64.77 10.06,64.77 | v13.79,23.7 13.79,22.45 | v13.61,40.06 13.44,40.06 | 39.22,94.28 39.22,84.51 SE_JK8.16 | 39.22,94.28 40.64,95.71 SE_AN1.14 | v28.91,99.09 28.02,99.09 25.53,96.6 25.53,95.88 SE_JK10.16 | v26.78,105.37 25.97,105.37 25.4,105.94 SE_JK11.16 | 39.22,94.28 37.62,94.28 34.42,97.49 v28.91,97.49 | v28.55,19.61 27.84,20.32 25.88,20.32 25.53,19.96 25.53,18.01 SE_N01.1 | v28.73,65.13 28.37,65.13 25.53,62.28 25.53,61.57 SE_JK3.16 | v27.66,74.55 26.42,74.55 25.53,73.66 25.53,72.95 SE_JK4.16 | v28.73,86.11 26.59,86.11 25.53,85.04 25.53,84.51 SE_JK9.16 | 53.26,51.79 53.26,51.97 50.6,54.63 50.6,59.79 52.2,61.39 53.26,61.39 BR_AA3.14 | 53.26,51.79 53.26,50.19 BR_AA2.14 53.26,50.01 51.49,50.01 47.93,46.46 39.22,46.46 38.86,46.1 | 29.62,40.59 34.24,40.59 35.48,39.34 | 29.62,40.59 27.48,40.59 25.53,42.55 25.53,45.57 26.59,46.63 26.59,50.01 BR_OR1.14 | M_OR1.14 35.48,39.34 | 38.86,46.1 38.33,45.57 38.33,42.19 35.48,39.34 | v41.71,26.37 39.75,26.37 38.86,25.48 38.86,24.77 PL_XR.14 | v38.51,48.59 39.22,49.3 39.22,50.01 BR_AA1.14 | SE_AN2.14 40.64,107.8 41.71,108.86 v42.42,108.86
  Top 0.152: BR_AA4.14 39.39,61.57 39.39,66.73 BR_NO4.1 39.39,66.9 39.39,67.44 40.46,68.5 v42.77,68.5 | v38.68,46.28 38.86,46.1 | 29.62,40.59 v29.62,40.95 | 25.88,36.86 27.66,38.63 v29.62,38.63 | PC_JK1.10 100.2,107.26 99.14,107.26 PC_JK1.11 98.96,107.26 98.96,107.97 97.89,109.04 93.27,109.04 | 93.27,109.04 88.29,109.04 87.4,108.15 85.27,108.15 84.56,108.86 | 84.56,108.86 84.56,109.93 86.33,111.71 M48Z08.28 | 62.51,112.06 62.51,112.95 63.4,113.84 SP_BF0.5 | 62.51,112.06 62.51,110.47 63.4,109.58 63.4,109.04 SP_BF1.5 | 55.22,112.06 55.22,112.6 54.15,113.66 54.15,114.73 55.22,115.8 SE_BF0.5 | 55.22,112.06 v55.22,111.89 55.22,110.82 SE_BF1.5 | 55.22,112.06 62.51,112.06 | 55.22,92.33 55.22,90.55 SE_BF5.5 | 55.22,92.33 54.15,93.4 54.15,94.46 55.22,95.53 SE_BF4.5 55.4,95.71 58.06,95.71 59.49,97.13 61.8,97.13 63.4,98.73 SP_BF3.5 63.58,98.91 63.58,99.26 64.47,100.15 64.47,102.82 63.58,103.71 SP_BF2.5 63.4,103.71 61.44,103.71 60.2,102.46 55.22,102.46 | 55.22,92.33 60.38,92.33 61.62,93.57 63.4,93.57 SP_BF4.5 | 55.22,102.46 55.22,100.69 SE_BF3.5 | 55.22,102.46 54.15,103.53 54.15,104.6 55.22,105.66 SE_BF2.5 55.4,105.84 55.57,106.02 58.78,106.02 61.62,108.86 63.4,108.86 SP_BF1.5 | 84.56,108.86 73,108.86 72.11,107.97 65.89,107.97 | 65.89,107.97 64.47,107.97 63.58,108.86 SP_BF1.5 | 57.71,77.93 57.53,77.75 54.51,77.75 54.15,78.1 54.15,79.17 55.22,80.24 SE_BF7.5 55.22,80.42 55.22,81.13 v54.69,81.66 | 57.71,77.93 58.06,78.28 63.4,78.28 SP_BF7.5 | 57.71,77.93 57.71,75.79 57.35,75.44 55.22,75.44 53.44,73.66 53.44,72.95 BR_OR2.14 | SP_BF5.5 63.4,88.42 60.2,88.42 57.35,85.57 55.4,85.57 SE_BF6.5 55.22,85.57 v55.22,86.46
  Top 0.152: 90.07,51.79 90.42,51.79 92.02,50.19 92.56,50.19 BR_JK2.16 | 90.07,51.79 v83.49,51.79 81.18,51.79 80.11,50.72 80.11,50.19 BR_JK1.16 | 90.07,51.79 92.56,54.28 92.56,55.35 BR_NO1.1 | v83.13,68.5 80.11,71.53 80.11,72.77 PC_AN2.14 | BR_NO2.1 67.31,33.12 69.27,35.08 76.91,35.08 79.22,32.77 79.22,30.45 79.93,29.74 v82.96,29.74 | v81.18,36.86 80.11,37.92 80.11,38.63 BR_JK5.16 | T1.B1 70.69,5.56 70.33,5.56 +5V.1 68.56,3.96 62.69,3.96 62.33,4.32 CLKNO.14 62.33,4.5 61.09,5.74 61.09,12.85 60.2,13.74 57,13.74 55.04,15.7 52.91,15.7 50.95,17.65 50.95,18.36 M_NO1.1 | v64.64,82.19 64.64,82.37 63.58,83.44 SP_BF6.5 | BR_AN1.14 67.31,50.72 65,53.04 65,58.55 66.42,59.97 | 66.42,59.97 67.31,60.86 BR_AN5.14 | 70.16,58.73 67.67,58.73 66.42,59.97 | 70.16,58.73 74.07,58.73 76.73,61.39 79.93,61.39 BR_OR5.14 | BR_OR4.14 67.31,25.3 69.98,27.96 70.51,27.96 | 70.51,27.96 78.51,27.96 79.22,27.25 | 79.22,27.25 79.93,26.54 79.93,24.77 BR_AN3.14 | BR_AN6.14 67.31,72.24 68.38,71.17 v69.27,71.17 | v70.51,27.61 70.51,27.96 | v70.16,56.95 70.16,58.73 | v82.96,27.43 81.18,27.43 80.64,27.96 79.93,27.96 79.22,27.25 | v65.89,107.26 65.89,107.97 | v56.29,51.79 53.26,51.79 | 93.27,109.04 v93.27,109.4
  Bottom 0.152: 96.29,94.11 v96.29,97.66 v96.29,99.44 96.29,104.06 C79.1 96.11,104.24 94.51,104.24 v93.27,105.49 v93.27,109.4 | 96.29,94.11 96.29,92.86 C19.1 96.29,92.69 96.29,86.28 v96.11,86.11 96.11,81.31 C49.1 96.11,81.13 96.11,70.46 | 96.29,94.11 v95.76,94.11 | v94.87,22.99 94.87,21.74 C6.1 95.05,21.74 96.11,22.81 96.11,35.43 C74.1 96.11,35.61 95.58,36.14 C75.1 | C75.1 96.11,47.52 96.11,58.37 C48.1 96.11,58.55 96.11,70.46 | 96.11,70.46 95.58,69.93 C50.1 | v94.51,71.17 95.4,70.28 95.4,69.93 C50.1 | 96.11,70.46 C50.1 | C75.1 | C34.1 110.16,21.74 v110.16,28.85 110.16,35.43 C80.1 110.16,35.61 v110.16,40.23 C95.1 | C95.1 v110.16,52.5 110.69,53.04 110.69,58.37 C7.1 110.69,58.55 110.52,58.73 v110.52,63.17 v110.52,65.13 110.52,69.57 110.34,69.75 C76.1 110.16,69.93 110.16,81.13 C51.1 110.16,81.31 110.16,92.69 C20.1 110.16,92.86 v110.16,97.49 v110.16,99.44 110.16,104.06 C30.1 | C95.1 | v126.34,105.49 126.16,105.31 126.16,104.24 C29.1 126.16,104.06 126.16,92.86 C23.1 125.98,92.69 v125.98,91.26 125.98,81.31 C22.1 125.98,81.13 125.98,71.35 | C78.1 122.25,21.74 122.78,22.28 122.78,33.48 125.98,36.68 C77.1 126.16,36.86 v126.16,38.28 126.16,48.23 C8.1 126.16,48.41 126.16,49.66 | 125.98,71.35 125.98,69.93 C21.1 125.98,69.75 125.98,60.5 | 126.16,49.66 126.16,58.37 C54.1 125.98,58.55 125.98,60.5 | 126.16,49.66 v125.45,49.66 | v122.78,59.79 123.5,60.5 125.98,60.5 | 125.98,71.35 v126.34,71.35 | C64.1 133.45,10.54 v134.52,11.61 134.52,14.45 | 134.52,14.45 133.45,15.52 C90.1 | 134.52,19.79 134.16,19.79 133.45,20.5 C41.1 | 134.52,14.45 v134.52,17.12 134.52,19.79 | 134.52,19.79 134.52,24.59 133.45,25.65 C65.1
  Bottom 0.152: 144.83,14.45 144.83,11.61 145.9,10.54 C91.1 | 144.83,14.45 145.9,15.52 C92.1 | 144.83,19.43 145.9,20.5 C66.1 | 144.83,14.45 144.83,19.43 | 144.83,24.59 144.65,24.41 144.65,19.61 144.83,19.43 | 144.83,24.59 145.9,25.65 C42.1 | 144.83,24.59 v144.83,26.72 140.03,31.52 140.03,36.68 C52.1 140.03,36.86 v140.03,41.66 140.03,48.23 C53.1 139.85,48.41 139.85,49.48 | v138.79,105.49 139.85,104.42 139.85,104.24 C28.1 140.03,104.06 v140.03,94.11 140.03,92.86 C24.1 139.85,92.69 139.68,92.51 139.68,90.91 139.85,90.73 v139.85,86.11 139.85,81.31 C25.1 140.03,81.13 140.03,70.46 140.56,69.93 C26.1 140.74,69.75 v140.74,65.13 140.74,58.55 C27.1 140.56,58.37 139.85,57.66 139.85,49.48 | 139.85,49.48 v139.68,49.66 | v13.44,105.49 13.61,105.31 13.61,104.24 C17.1 13.61,104.06 v13.61,98.73 13.61,92.86 C18.1 13.61,92.69 13.61,81.31 C81.1 13.61,81.13 v13.61,76.15 13.61,69.93 C32.1 13.61,69.75 v13.61,64.77 13.61,58.55 C15.1 13.61,58.37 13.61,46.99 | C10.2 13.97,22.63 13.79,22.81 v13.79,23.7 13.79,32.94 C14.1 | 13.61,33.48 v12.72,34.37 | 13.61,33.48 13.61,33.12 C14.1 | 13.61,46.99 v13.61,40.06 13.61,33.48 | 13.61,33.48 C14.1 | 13.61,46.99 C35.1 | v26.78,105.37 28.02,104.14 C55.1 28.91,104.06 v28.91,99.09 v28.91,97.49 28.91,92.86 C56.1 28.73,92.69 v28.73,86.11 28.73,81.31 C31.1 28.91,81.13 28.91,74.55 | v28.55,19.61 28.73,19.79 28.73,20.85 C13.1 28.91,21.03 29.44,21.57 29.44,32.94 C16.1 29.62,33.12 v29.62,38.63 v29.62,40.95 29.62,46.99 C94.1 29.44,46.99 28.91,47.52 28.91,58.37 C84.1 28.73,58.55 v28.73,65.13 28.73,69.75 C33.1 28.91,69.93 28.91,74.55 | 28.91,74.55 v27.66,74.55
  Bottom 0.152: C3.1 41.71,21.74 v41.71,26.37 41.71,32.94 C72.1 41.71,33.12 41.71,44.86 | v38.51,48.59 38.68,48.41 v38.68,46.28 38.68,45.21 39.04,44.86 41.71,44.86 | 41.71,44.86 42.06,44.86 42.06,46.99 C67.1 42.24,58.37 C68.1 42.24,58.55 42.24,67.97 v42.77,68.5 42.77,69.75 C43.1 42.95,69.93 42.95,81.13 C57.1 42.95,81.31 43.31,81.66 43.31,92.51 43.48,92.69 C83.1 43.48,92.86 43.48,104.06 C82.1 43.48,104.24 43.48,107.8 v42.42,108.86 | C93.1 56.29,46.99 v56.29,51.79 56.29,58.37 C11.1 56.29,58.55 57,59.26 57,69.04 56.29,69.75 C69.1 56.11,69.93 55.57,70.46 55.57,81.31 55.22,81.66 | 55.22,81.66 54.69,81.13 | 54.69,81.13 53.98,80.42 C59.1 | 55.22,84.15 55.22,81.66 | 55.22,84.15 53.98,85.4 C60.1 | 55.22,89.66 54.69,89.66 53.98,90.37 C61.1 | 55.22,84.15 v55.22,86.46 55.22,89.66 | 55.22,94.82 54.69,94.82 53.98,95.53 C88.1 | 55.22,89.66 55.22,94.82 | 55.22,99.8 54.69,99.8 53.98,100.51 C62.1 | 55.22,94.82 55.22,99.8 | 55.22,104.95 54.69,104.95 53.98,105.66 C63.1 | 55.22,99.8 55.22,104.95 | 55.22,109.93 54.69,109.93 53.98,110.64 C89.1 | 55.22,104.95 55.22,109.93 | 55.22,109.93 v55.22,111.89 55.22,115.09 54.69,115.09 53.98,115.8 C86.1 | 54.69,81.13 v54.69,81.66 | 82.96,68.5 82.96,58.55 C2.1 82.96,58.37 83.49,57.84 v83.49,51.79 C45.1 | 82.96,68.5 82.96,69.75 C71.1 | 82.96,68.5 v83.13,68.5 | C5.1 82.96,21.74 v82.96,27.43 v82.96,29.74 82.96,34.9 83.49,35.43 C47.1 83.49,35.61 83.49,37.57 | 83.49,37.57 C45.1 | v81.18,36.86 81.89,37.57 83.49,37.57 | C45.1 | C4.1 54.33,21.57 54.33,17.65 55.75,16.23 55.75,8.76 56.11,8.41 C12.1 56.29,8.23 58.42,6.1 62.15,6.1 62.15,4.5 CLKNO.14 | v64.64,82.19 64.64,83.44 C40.1 64.82,83.44 65.89,82.37
  Bottom 0.152: 66.24,79.88 64.82,78.46 C36.1 | 66.24,79.88 66.24,82.02 65.89,82.37 | 65.89,87.35 64.82,88.42 C39.1 | 65.89,82.37 65.89,87.35 | 65.89,92.51 64.82,93.57 C38.1 | 65.89,87.35 65.89,92.51 | 65.89,97.66 64.82,98.73 C37.1 | 65.89,92.51 65.89,97.66 | 65.89,102.64 64.82,103.71 C58.1 | 65.89,97.66 65.89,102.64 | 65.89,107.8 64.82,108.86 C87.1 | 65.89,102.64 v65.89,107.26 65.89,107.8 | 65.89,107.8 65.89,112.78 64.82,113.84 C85.1 | 70.69,27.61 70.69,35.43 C46.1 70.87,35.61 70.87,44.68 70.33,45.21 70.33,46.99 C1.1 70.16,46.99 v70.16,56.95 70.16,58.37 C70.1 70.16,58.55 70.16,69.75 C44.1 70.16,69.93 70.16,70.28 v69.27,71.17 69.27,76.86 66.24,79.88 | 70.69,27.61 70.69,22.1 70.33,21.74 C73.1 70.16,21.57 69.8,21.21 69.8,6.63 70.69,5.74 T1.B1 | 70.69,27.61 v70.51,27.61
BR_CM_N0  (via drill 0.35)
  Top 0.152: v83.67,26.37 83.67,24.77 BR_AN3.11
  Route15 0.152: v83.67,26.37 83.67,25.83 86.16,23.34 86.16,8.05 COM.1
BR_CM_N1
  Top 0.152: BR_AN3.10 85.09,26.37 83.13,28.32 67.49,28.32 66.6,27.43 66.6,16.59 69.98,13.21 75.13,13.21 84.38,3.96 COM.2
BR_CM_N2  (via drill 0.35)
  Top 0.152: v54.86,70.99 55.93,70.99 57,72.06 57,72.77 BR_OR2.11 | v54.33,14.1 54.69,14.1 56.11,12.68 56.11,10.19 61.09,5.21 61.09,3.43 61.8,2.72 69.44,2.72 71.93,5.21 71.93,6.1 69.09,8.94 67.49,8.94 67.13,9.3 67.13,10.01 67.49,10.36 71.4,10.36 75.67,6.1 77.27,6.1 81.53,1.83 84.91,1.83 86.87,3.79 COM.3
  Bottom 0.152: v54.86,70.99 54.86,24.05 53.26,22.45 53.26,15.16 v54.33,14.1
BR_CM_N3
  Top 0.152: COM.4 89.53,9.3 82.6,16.23 82.6,18.36 BR_AN3.3
BR_NR_N0  (via drill 0.35)
  Top 0.152: v72.82,20.14 71.22,21.74 71.22,24.59 BR_OR4.11
  Route15 0.152: v72.82,20.14 72.82,14.99 80.82,6.98 80.82,3.25 81.36,2.72 92.91,2.72 93.98,3.79 NU/AD.1
BR_NR_N1
  Top 0.152: BR_OR4.3 69.98,18.36 69.98,16.76 71.04,15.7 81,15.7 82.6,14.1 83.67,14.1 88.29,9.47 88.82,9.47 89.18,9.12 89.18,5.92 88.29,5.03 88.29,2.72 89.18,1.83 94.51,1.83 96.47,3.79 NU/AD.2
BR_NR_N2  (via drill 0.35)
  Top 0.152: v71.22,16.76 71.22,18.36 BR_OR4.4
  Route15 0.152: v71.22,16.76 71.22,14.1 80.47,4.85 80.47,3.07 81.18,2.36 97.54,2.36 98.96,3.79 NU/AD.3
BR_NR_N3  (via drill 0.35)
  Top 0.152: v72.82,22.99 72.47,23.34 72.47,24.59 BR_OR4.10
  Route15 0.152: v72.82,22.99 72.82,21.21 70.51,18.9 70.51,14.1 80.11,4.5 80.11,2.9 81,2.01 99.67,2.01 101.45,3.79 NU/AD.4
BR_READ  (via drill 0.35)
  Top 0.152: v61.8,47.7 60.73,46.63 57.35,46.63 54.69,49.3 54.69,50.01 BR_AA2.13 | 68.2,47.7 v65.35,47.7 | 68.2,47.7 69.8,49.3 69.8,50.01 BR_AN1.12 | v143.59,11.61 144.65,10.54 RE_BF0.1 | v143.59,15.34 144.48,15.34 144.65,15.52 RE_BF1.1 | v143.59,20.5 144.65,20.5 RE_BF2.1 | v143.41,25.48 143.59,25.65 144.65,25.65 RE_BF3.1 | 119.41,20.68 119.41,21.57 121.36,23.52 | 119.41,20.68 119.41,18.54 BR_AN2.1 | 121.36,23.52 121.89,24.05 121.89,24.59 BR_AN2.12 | 121.36,23.52 124.03,20.85 | 124.03,20.85 124.38,20.5 124.38,18.54 BR_AN2.5 | 124.03,20.85 126.87,23.7 126.87,24.59 BR_AN2.8 127.05,24.77 128.47,24.77 130.78,27.08 133.45,27.08 133.99,26.54 v142.34,26.54 | v68.38,47.7 68.2,47.7 | v67.84,9.65 70.69,9.65 74.6,5.74 77.09,5.74 81.71,1.12 113.89,1.12 117.45,4.67 117.45,11.07 v119.05,12.68 | 119.41,20.68 v119.05,20.68
  Route2 0.152: v65.35,47.7 v61.8,47.7 | v142.34,26.54 v143.41,25.48
  Bottom 0.152: v143.59,11.61 v143.59,15.34 v143.59,20.5 143.59,25.3 v143.41,25.48 | v68.38,47.7 68.38,19.07 67.84,18.54 v67.84,9.65 | v119.05,20.68 v119.05,12.68
BR_SET  (via drill 0.35)
  Top 0.152: BR_JK7.3 125.09,32.23 126.34,30.99 137.01,30.99 138.25,32.23 | 138.25,32.23 138.96,32.94 138.96,33.66 BR_JK8.3 | 126.52,40.95 126.52,40.06 BR_JK7.13 | 126.52,40.95 127.58,42.01 131.5,42.01 133.63,39.88 133.63,39.52 135.41,37.74 138.43,37.74 | 138.43,37.74 138.79,37.74 140.21,39.17 140.21,39.88 BR_JK8.13 | v138.43,32.05 138.25,32.23 | 138.43,37.74 v138.43,38.28 | M_OR1.9 45.09,34.19 v45.97,33.3 | v98.42,15.7 99.49,15.7 100.56,16.76 106.6,16.76 | 106.6,16.76 108.74,16.76 109.8,17.83 109.8,18.36 BR_AN7.3 109.98,18.54 109.98,20.14 111.05,21.21 111.05,24.59 BR_AN7.11 | 126.52,40.95 125.98,40.95 124.92,42.01 124.03,42.01 123.85,42.19 119.76,42.19 117.63,40.06 117.63,32.59 117.8,32.41 117.8,30.45 116.2,28.85 112.12,28.85 111.4,29.57 109.45,29.57 106.6,26.72 106.6,16.76
  Route2 0.152: v45.97,33.3 45.97,31.7 61.62,16.05 98.07,16.05 v98.42,15.7
  Bottom 0.152: v138.43,38.28 v138.43,32.05
BR_SET_N0
  Top 0.152: BR_JK3.1 122.43,45.21 122.43,49.48 121.89,50.01 121.89,56.06 123.5,57.66 127.41,57.66 128.12,56.95 128.12,55.35 PC_AN1.5
BR_SET_N1
  Top 0.152: PC_AN1.1 123.32,55.35 123.32,51.79 123.67,51.44 BR_JK3.15
BR_SET_N2
  Top 0.152: PC_AN1.8 130.78,61.39 130.78,57.3 135.76,52.32 135.76,45.92 136.47,45.21 BR_JK4.1
BR_SET_N3
  Top 0.152: PC_AN1.12 125.81,61.57 125.81,62.28 127.05,63.52 132.92,63.52 134.34,62.1 134.34,59.61 135.41,58.55 146.61,58.55 147.5,57.66 147.5,54.28 146.25,53.04 138.79,53.04 137.9,52.15 137.9,51.44 BR_JK4.15
BR_SET_N4
  Top 0.152: BR_JK5.1 79.93,32.59 77.09,35.43 68.56,35.43 64.29,39.7 64.29,63.88 65.35,64.95 65.35,66.73 68.38,69.75 76.02,69.75 78.87,66.9 79.93,66.9 PC_AN2.1
BR_SET_N5  (via drill 0.35)
  Top 0.152: v78.69,41.12 79.4,41.12 81.18,39.34 81.18,38.63 BR_JK5.15 | v79.22,65.3 84.2,65.3 85.09,66.19 PC_AN2.5
  Bottom 0.152: v78.69,41.12 78.51,41.3 78.51,64.59 v79.22,65.3
BR_SET_N6  (via drill 0.35)
  Top 0.152: v89.71,71.35 88.29,72.77 87.76,72.77 PC_AN2.8 | v89.89,43.08 90.42,42.55 90.42,39.34 91.49,38.28 91.49,35.79 92.56,34.72 92.56,32.59 BR_JK6.1
  Bottom 0.152: v89.71,71.35 89.36,70.99 89.36,43.61 v89.89,43.08
BR_SET_N7
  Top 0.152: BR_JK6.15 93.98,40.59 94.34,40.95 100.91,40.95 103.76,43.79 103.76,65.3 100.91,68.15 100.91,68.5 99.67,69.75 93.27,69.75 92.38,70.64 84.2,70.64 82.6,72.24 82.6,72.77 PC_AN2.12
BR_SET_N8
  Top 0.152: BR_JK1.1 79.93,43.97 79.93,44.32 78.51,45.75 78.51,50.9 79.93,52.32 82.42,52.32 82.6,52.5 87.22,52.5 90.78,56.06 90.78,64.95 92.56,66.73 PC_AN3.1
BR_SET_N9  (via drill 0.35)
  Top 0.152: v119.76,36.5 122.43,33.83 BR_JK7.1 | v98.42,68.5 98.42,67.97 97.89,67.44 97.89,66.9 PC_AN3.5
  Route2 0.152: v119.23,68.68 117.63,68.68 116.03,70.28 100.2,70.28 v98.42,68.5
  Bottom 0.152: v119.76,36.5 119.23,37.03 v119.23,68.68
BR_SET_N10  (via drill 0.35)
  Top 0.152: v119.94,41.3 123.14,41.3 123.67,40.77 123.67,40.06 BR_JK7.15 | v103.23,72.41 100.74,72.41 100.38,72.77 PC_AN3.8
  Route2 0.152: v119.58,71.88 119.41,71.7 108.03,71.7 107.31,72.41 v103.23,72.41
  Bottom 0.152: v119.94,41.3 119.94,71.53 v119.58,71.88
BR_SET_N11  (via drill 0.35)
  Top 0.152: v94.69,74.55 95.22,74.02 95.22,72.95 PC_AN3.12 | v132.56,31.7 134.52,31.7 136.47,33.66 BR_JK8.1
  Route2 0.152: v95.4,30.81 98.25,27.96 100.38,27.96 103.4,24.94 105.36,24.94 110.34,19.96 110.34,19.79 110.69,19.43 116.2,19.43 122.43,25.65 126.52,25.65 v132.56,31.7
  Bottom 0.152: v94.69,74.55 93.45,73.3 93.45,48.95 93.8,48.59 93.8,37.92 95.22,36.5 95.22,30.99 v95.4,30.81
BR_SET_N12
  Top 0.152: BR_JK8.15 137.72,39.88 137.72,39.17 137.01,38.46 135.59,38.46 131.67,42.37 124.21,42.37 124.03,42.55 122.43,42.55 118.16,46.81 118.16,52.86 117.09,53.92 117.09,56.24 114.25,59.08 112.29,59.08 110.52,60.86 110.52,61.39 PC_AN4.12
GND  (via drill 0.35)  (1 unrouted)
